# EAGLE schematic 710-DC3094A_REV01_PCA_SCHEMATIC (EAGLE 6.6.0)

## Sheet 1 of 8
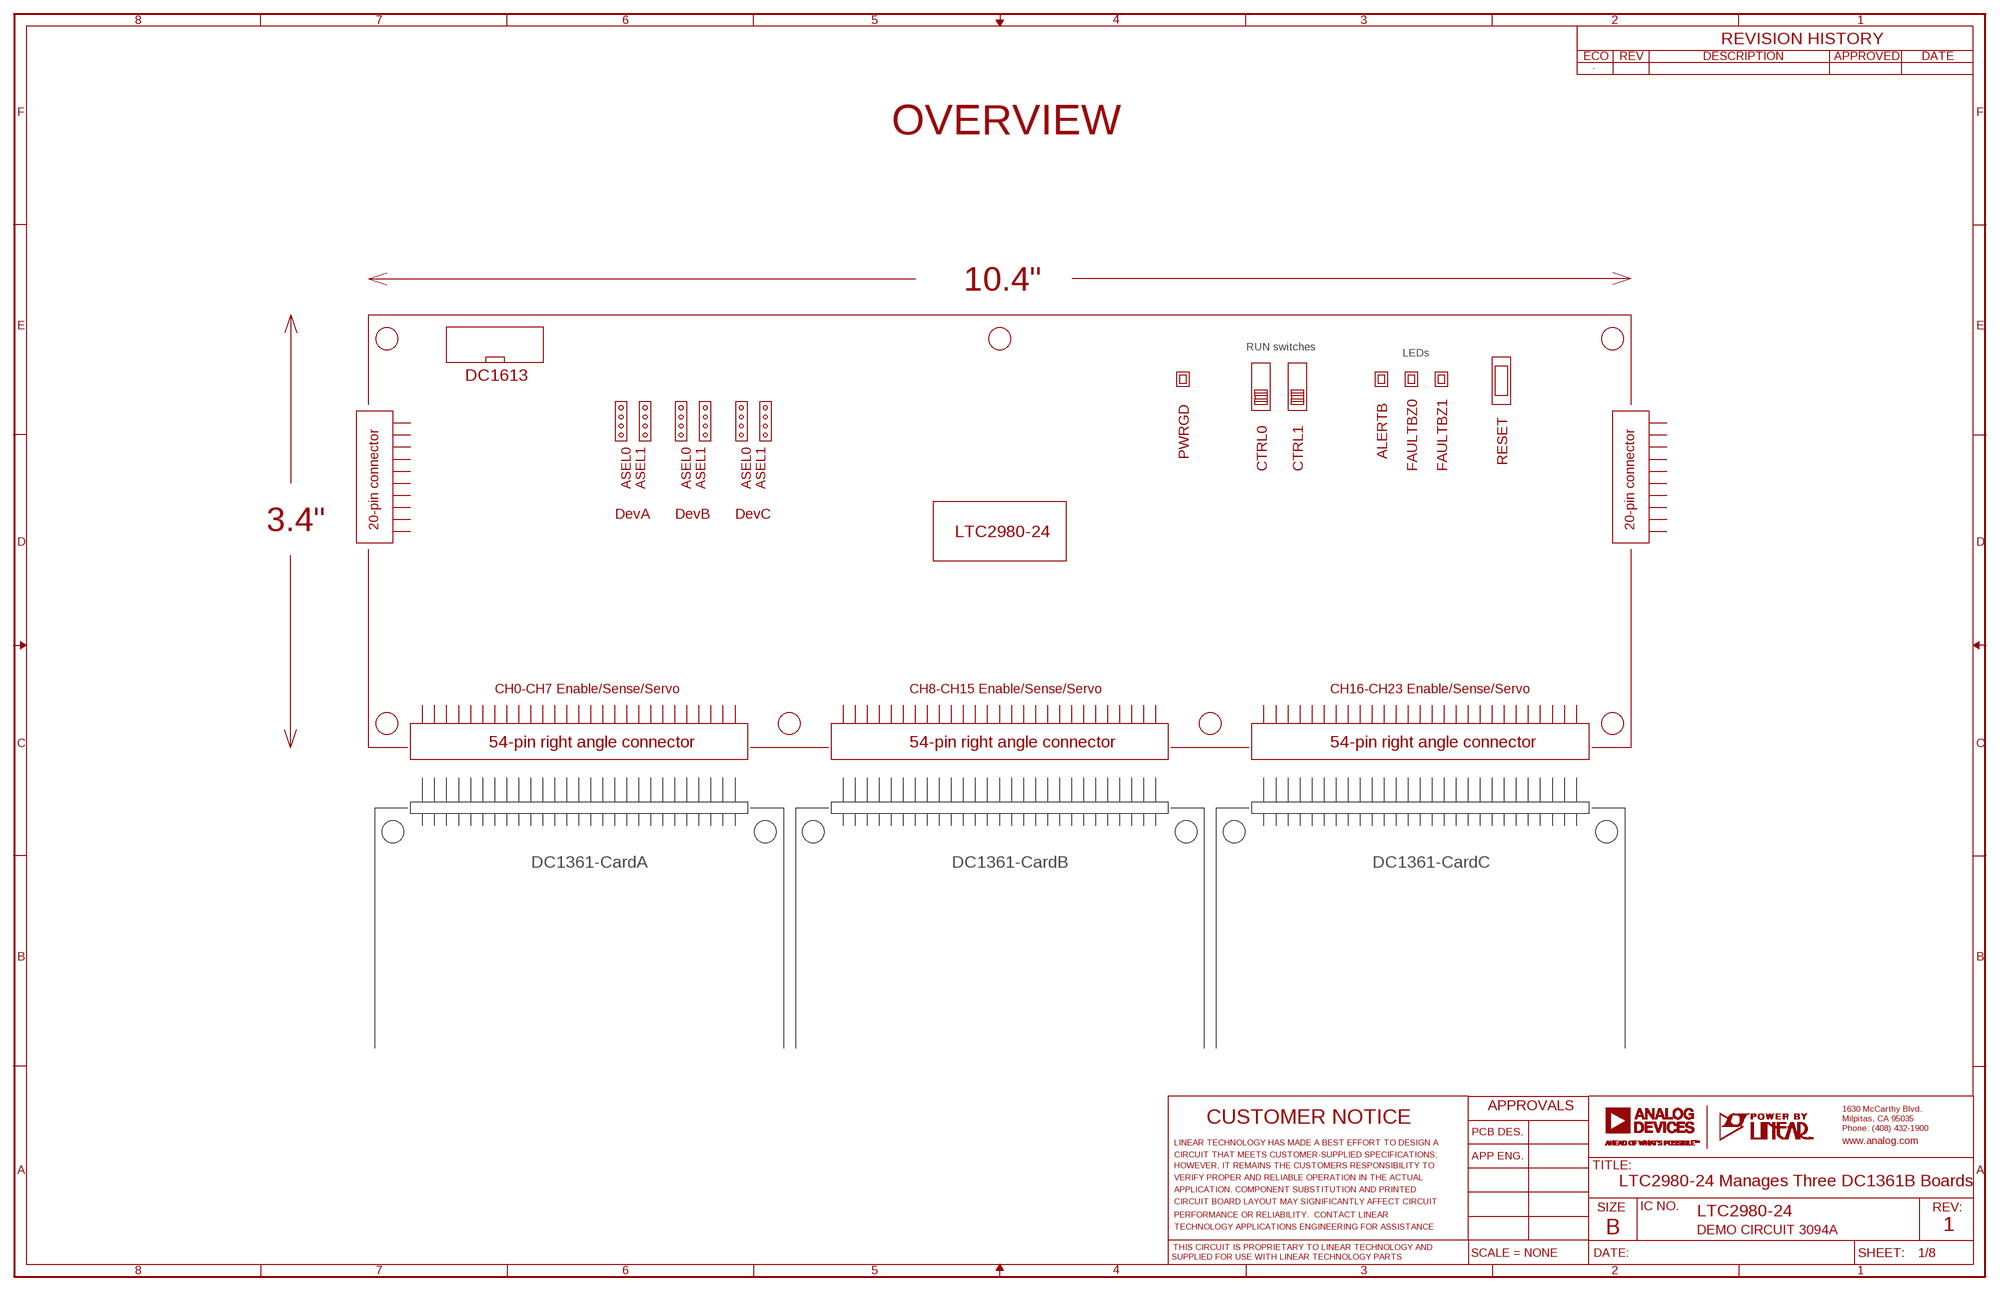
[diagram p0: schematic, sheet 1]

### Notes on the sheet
- OVERVIEW
- 10.4"
- RUN switches
- LEDs
- DC1613
- 20-pin connector | 20-pin connector
- ASEL0
  ASEL1
- ASEL0
  ASEL1
- ASEL0
  ASEL1
- PWRGD | ALERTB
- RESET
- CTRL0 | CTRL1 | FAULTBZ0 | FAULTBZ1
- DevA | DevB | DevC
- 3.4"
- LTC2980-24
- CH0-CH7 Enable/Sense/Servo | CH8-CH15 Enable/Sense/Servo | CH16-CH23 Enable/Sense/Servo
- 54-pin right angle connector | 54-pin right angle connector | 54-pin right angle connector
- DC1361-CardA | DC1361-CardB | DC1361-CardC
- LTC2980-24 Manages Three DC1361B Boards
- LTC2980-24
- DEMO CIRCUIT 3094A | 1

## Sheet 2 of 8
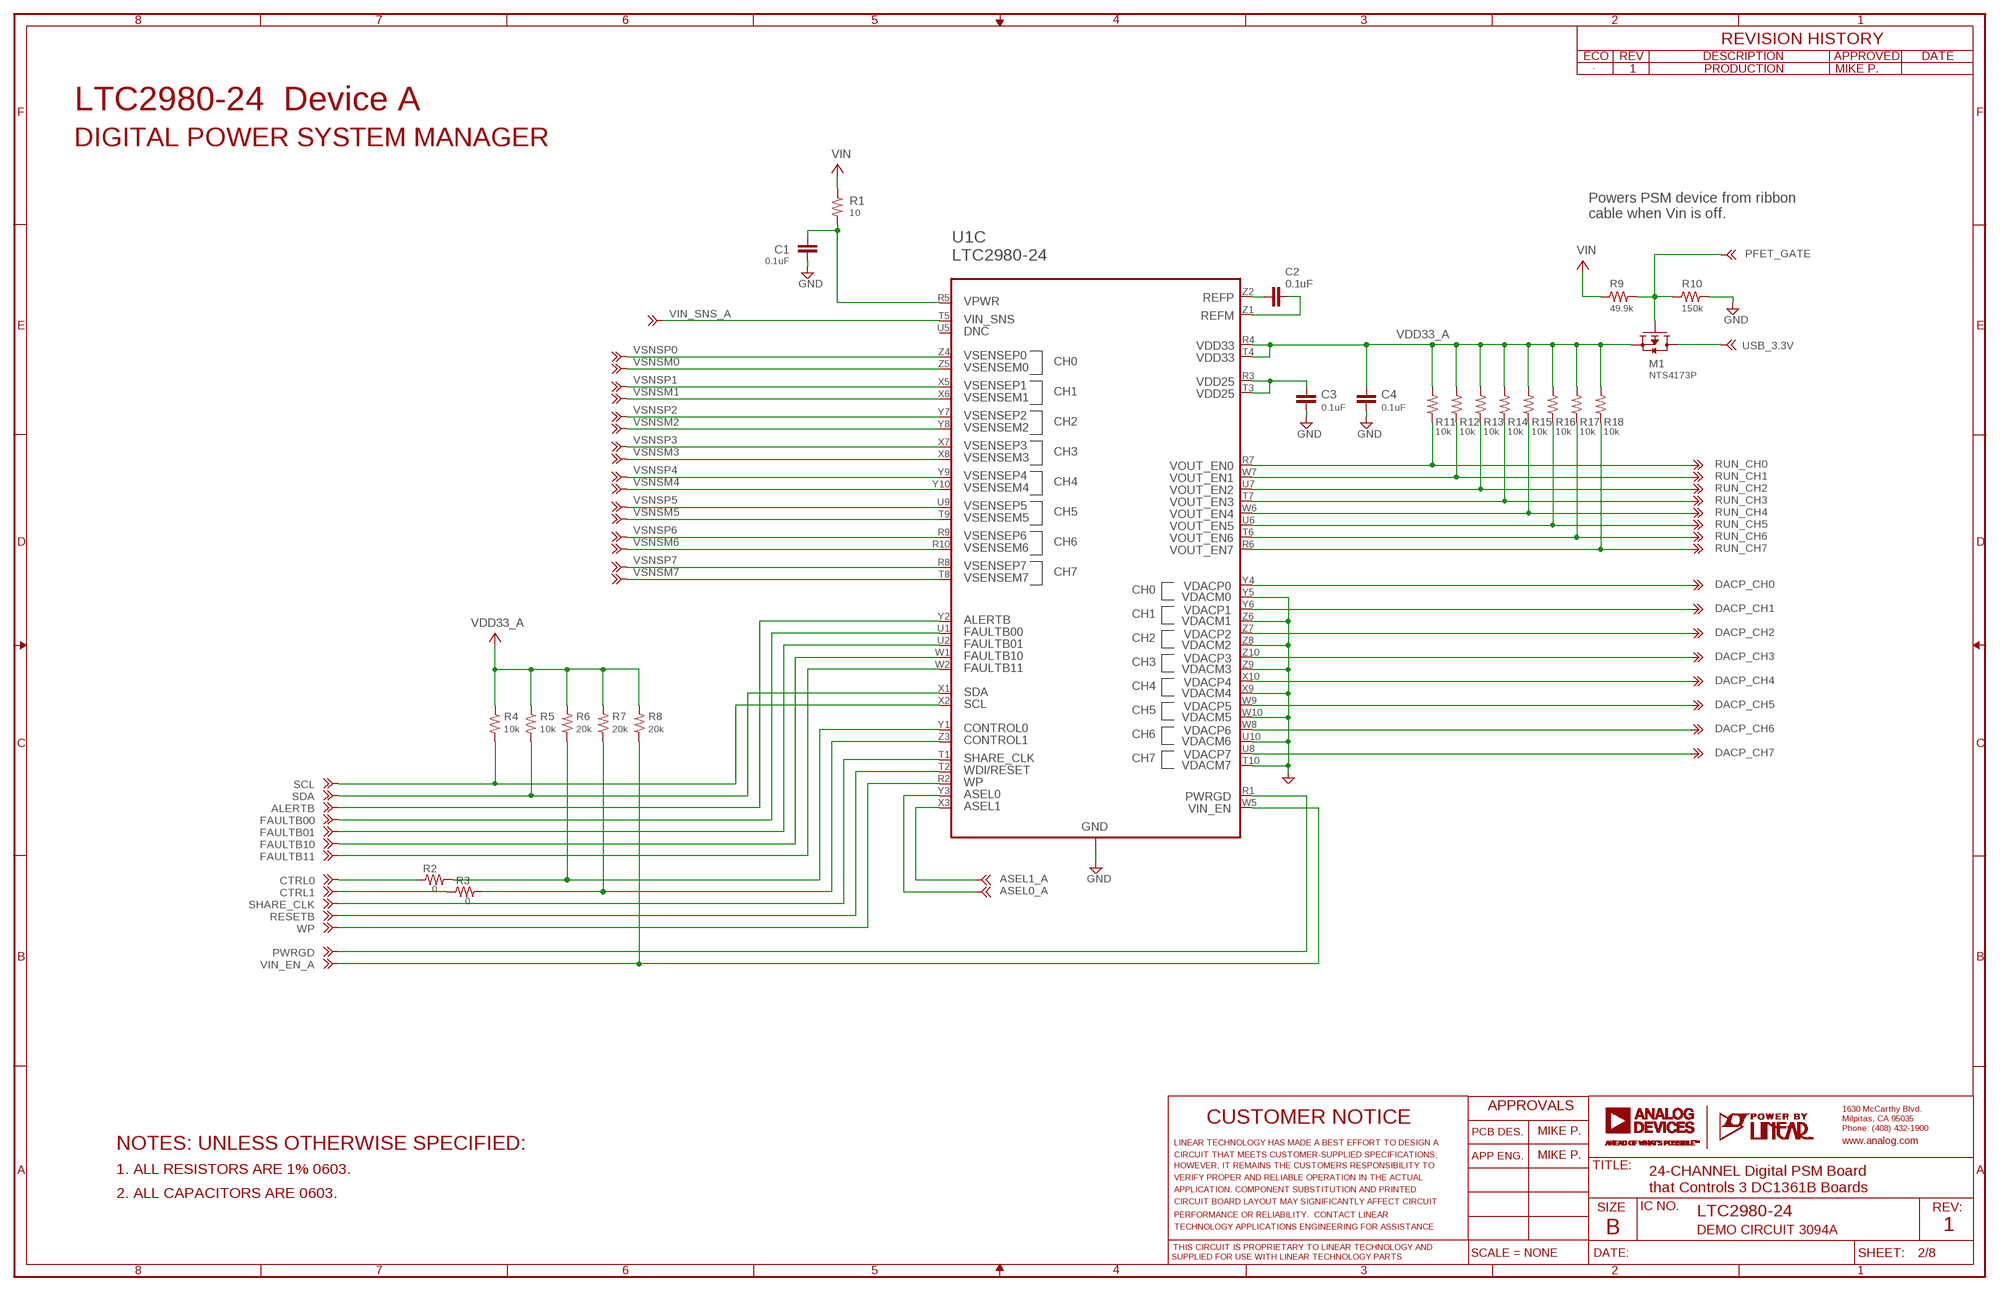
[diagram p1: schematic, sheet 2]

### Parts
C1  0.1uF  CC0603_BOX  [C0603_BOX]
C2  0.1uF  CC0603_BOX  [C0603_BOX]
C3  0.1uF  CC0603_BOX  [C0603_BOX]
C4  0.1uF  CC0603_BOX  [C0603_BOX]
M1  NTS4173P  PCH_SOT323  [SOT323@1]
R1  10  RR0603_BOX  [R0603_BOX]
R2  0  RR0603_BOX  [R0603_BOX]
R3  0  RR0603_BOX  [R0603_BOX]
R4  10k  RR0603_BOX  [R0603_BOX]
R5  10k  RR0603_BOX  [R0603_BOX]
R6  20k  RR0603_BOX  [R0603_BOX]
R7  20k  RR0603_BOX  [R0603_BOX]
R8  20k  RR0603_BOX  [R0603_BOX]
R9  49.9k  RR0402_BOX  [R0402_BOX]
R10  150k  RR0402_BOX  [R0402_BOX]
R11  10k  RR0603_BOX  [R0603_BOX]
R12  10k  RR0603_BOX  [R0603_BOX]
R13  10k  RR0603_BOX  [R0603_BOX]
R14  10k  RR0603_BOX  [R0603_BOX]
R15  10k  RR0603_BOX  [R0603_BOX]
R16  10k  RR0603_BOX  [R0603_BOX]
R17  10k  RR0603_BOX  [R0603_BOX]
R18  10k  RR0603_BOX  [R0603_BOX]
U1  LTC2980-24  LTC2980-24X  [BGA210]

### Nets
ALERTB: U1.Y2(C:ALERT) ; also sheet 3,4,5,8
ASEL0_A: U1.Y3(C:ASEL0) ; also sheet 5
ASEL1_A: U1.X3(C:ASEL1) ; also sheet 5
CTRL0: R2.1 ; also sheet 3,4,5,8
CTRL0_C: R2.2 R6.1 U1.Y1(C:CTRL0)
CTRL1: R3.1 ; also sheet 3,4,5,8
CTRL1_C: R3.2 R7.1 U1.Z3(C:CTRL1)
DACP_CH0: U1.Y4(C:DACP0) ; also sheet 7
DACP_CH1: U1.Y6(C:DACP1) ; also sheet 7
DACP_CH2: U1.Z7(C:DACP2) ; also sheet 7
DACP_CH3: U1.Z10(C:DACP3) ; also sheet 7
DACP_CH4: U1.X10(C:DACP4) ; also sheet 7
DACP_CH5: U1.W9(C:DACP5) ; also sheet 7
DACP_CH6: U1.W8(C:DACP6) ; also sheet 7
DACP_CH7: U1.U8(C:DACP7) ; also sheet 7
FAULTB00: U1.U1(C:FLT00) ; also sheet 3,4,5,8
FAULTB01: U1.U2(C:FLT01) ; also sheet 3,4,5,8
FAULTB10: U1.W1(C:FLT10) ; also sheet 3,4,5,8
FAULTB11: U1.W2(C:FLT11) ; also sheet 3,4,5,8
GND: C1.2 C3.2 C4.2 R10.2 U1.T10(C:DACM7) U1.U3(C:GND) U1.U4(C:GND) U1.U10(C:DACM6) U1.W3(C:GND) U1.W4(C:GND) U1.W10(C:DACM5) U1.X4(C:GND) U1.X9(C:DACM4) U1.Y5(C:DACM0) U1.Z6(C:DACM1) U1.Z8(C:DACM2) U1.Z9(C:DACM3) ; also sheet 3,4,5,6,7,8
PFET_GATE: M1.1(G) R9.2 R10.1 ; also sheet 3,4
PWRGD: U1.R1(C:PWRGD) ; also sheet 3,4,5
REFM_C: C2.2 U1.Z1(C:REFM)
REFP_C: C2.1 U1.Z2(C:REFP)
RESETB: U1.T2(C:WDI) ; also sheet 3,4,5,8
RUN_CH0: R11.1 U1.R7(C:EN0) ; also sheet 7
RUN_CH1: R12.1 U1.W7(C:EN1) ; also sheet 7
RUN_CH2: R13.1 U1.U7(C:EN2) ; also sheet 7
RUN_CH3: R14.1 U1.T7(C:EN3) ; also sheet 7
RUN_CH4: R15.1 U1.W6(C:EN4) ; also sheet 7
RUN_CH5: R16.1 U1.U6(C:EN5) ; also sheet 7
RUN_CH6: R17.1 U1.T6(C:EN6) ; also sheet 7
RUN_CH7: R18.1 U1.R6(C:EN7) ; also sheet 7
SCL: R4.2 U1.X2(C:SCL) ; also sheet 3,4,8
SDA: R5.2 U1.X1(C:SDA) ; also sheet 3,4,8
SHARE_CLK: U1.T1(C:SHARE_CLK) ; also sheet 3,4,8
USB_3.3V: M1.3(D) ; also sheet 3,4,8
VDD25_C: C3.1 U1.R3(C:VDD25-IN) U1.T3(C:VDD25-OUT)
VDD33_A: C4.1 M1.2(S) R4.1 R5.1 R6.2 R7.2 R8.2 R11.2 R12.2 R13.2 R14.2 R15.2 R16.2 R17.2 R18.2 U1.R4(C:VDD33-IN) U1.T4(C:VDD33-OUT) ; also sheet 5
VIN: R1.1 R9.1 ; also sheet 3,4,7
VIN_A: C1.1 R1.2 U1.R5(C:VPWR)
VIN_EN_A: R8.1 U1.W5(C:VINEN) ; also sheet 7,8
VIN_SNS_A: U1.T5(C:VINSNS) ; also sheet 7,8
VSNSM0: U1.Z5(C:VSM0) ; also sheet 6
VSNSM1: U1.X6(C:VSM1) ; also sheet 6
VSNSM2: U1.Y8(C:VSM2) ; also sheet 6
VSNSM3: U1.X8(C:VSM3) ; also sheet 6
VSNSM4: U1.Y10(C:VSM4) ; also sheet 6
VSNSM5: U1.T9(C:VSM5) ; also sheet 6
VSNSM6: U1.R10(C:VSM6) ; also sheet 6
VSNSM7: U1.T8(C:VSM7) ; also sheet 6
VSNSP0: U1.Z4(C:VSP0) ; also sheet 6
VSNSP1: U1.X5(C:VSP1) ; also sheet 6
VSNSP2: U1.Y7(C:VSP2) ; also sheet 6
VSNSP3: U1.X7(C:VSP3) ; also sheet 6
VSNSP4: U1.Y9(C:VSP4) ; also sheet 6
VSNSP5: U1.U9(C:VSP5) ; also sheet 6
VSNSP6: U1.R9(C:VSP6) ; also sheet 6
VSNSP7: U1.R8(C:VSP7) ; also sheet 6
WP: U1.R2(C:WP) ; also sheet 3,4,5
Unconnected: U1.U5(C:DNC)

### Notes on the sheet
- 1 | PRODUCTION | MIKE P.
- LTC2980-24  Device A
- DIGITAL POWER SYSTEM MANAGER
- Powers PSM device from ribbon
  cable when Vin is off.
- MIKE P.
- NOTES: UNLESS OTHERWISE SPECIFIED:
- MIKE P.
- 1. ALL RESISTORS ARE 1% 0603.
- 24-CHANNEL Digital PSM Board
  that Controls 3 DC1361B Boards
- 2. ALL CAPACITORS ARE 0603.
- LTC2980-24
- DEMO CIRCUIT 3094A | 1

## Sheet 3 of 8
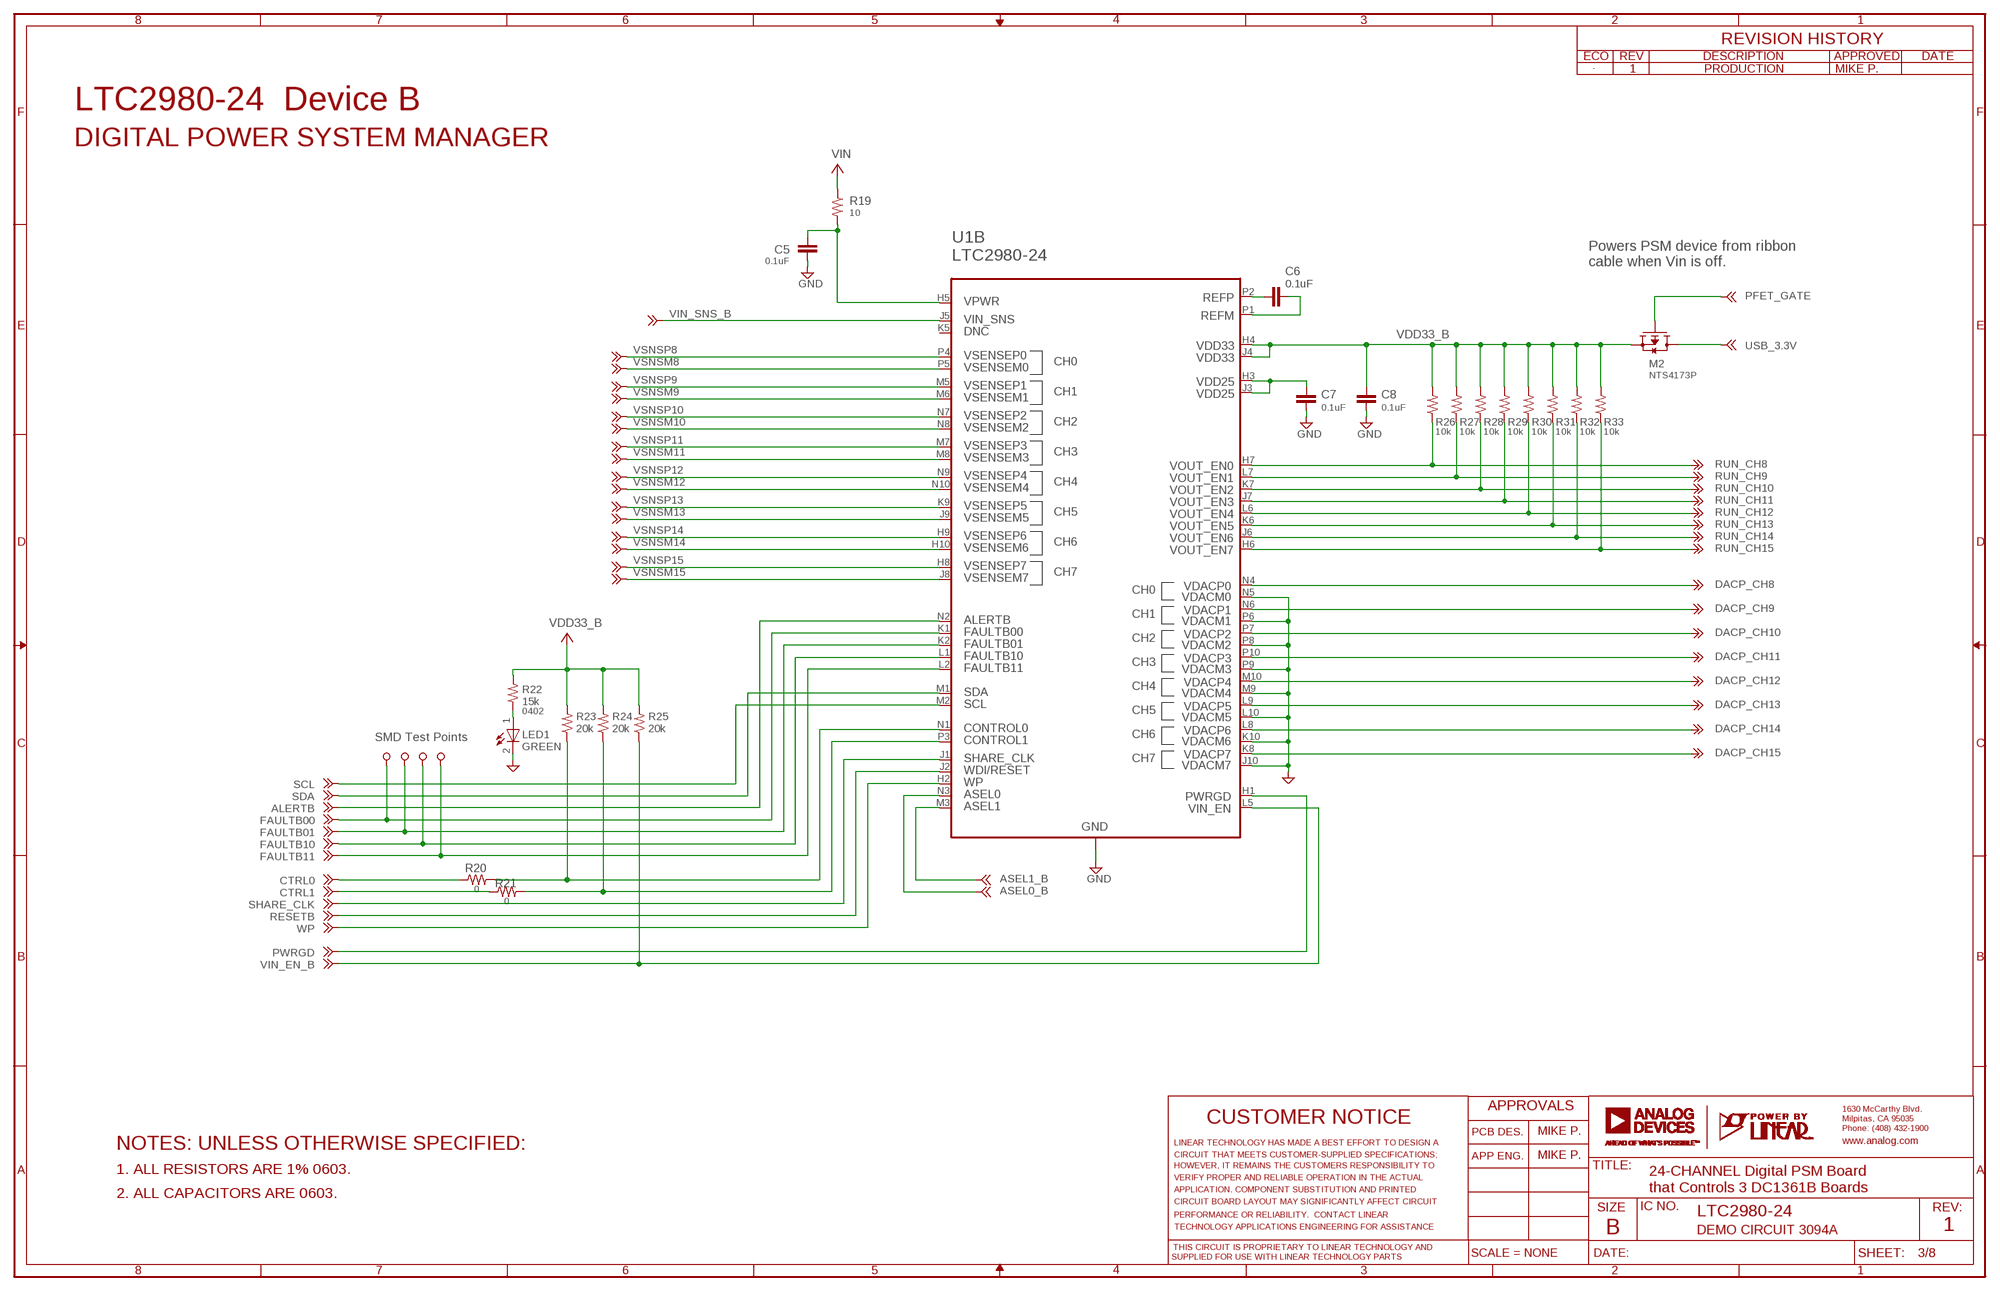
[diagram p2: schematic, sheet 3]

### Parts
C5  0.1uF  CC0603_BOX  [C0603_BOX]
C6  0.1uF  CC0603_BOX  [C0603_BOX]
C7  0.1uF  CC0603_BOX  [C0603_BOX]
C8  0.1uF  CC0603_BOX  [C0603_BOX]
LED1  GREEN  LED-0603  [CHIPLED_0603]
M2  NTS4173P  PCH_SOT323  [SOT323@1]
R19  10  RR0603_BOX  [R0603_BOX]
R20  0  RR0603_BOX  [R0603_BOX]
R21  0  RR0603_BOX  [R0603_BOX]
R22  15k  RR0402_BOX  [R0402_BOX]
R23  20k  RR0603_BOX  [R0603_BOX]
R24  20k  RR0603_BOX  [R0603_BOX]
R25  20k  RR0603_BOX  [R0603_BOX]
R26  10k  RR0603_BOX  [R0603_BOX]
R27  10k  RR0603_BOX  [R0603_BOX]
R28  10k  RR0603_BOX  [R0603_BOX]
R29  10k  RR0603_BOX  [R0603_BOX]
R30  10k  RR0603_BOX  [R0603_BOX]
R31  10k  RR0603_BOX  [R0603_BOX]
R32  10k  RR0603_BOX  [R0603_BOX]
R33  10k  RR0603_BOX  [R0603_BOX]
TP10  TESTPOINTVIA  [VIA]
TP11  TESTPOINTVIA  [VIA]
TP12  TESTPOINTVIA  [VIA]
TP13  TESTPOINTVIA  [VIA]

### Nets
ALERTB: U1.N2(B:ALERT) ; also sheet 2,4,5,8
ASEL0_B: U1.N3(B:ASEL0) ; also sheet 5
ASEL1_B: U1.M3(B:ASEL1) ; also sheet 5
CTRL0: R20.1 ; also sheet 2,4,5,8
CTRL0_B: R20.2 R23.1 U1.N1(B:CTRL0)
CTRL1: R21.1 ; also sheet 2,4,5,8
CTRL1_B: R21.2 R24.1 U1.P3(B:CTRL1)
DACP_CH8: U1.N4(B:DACP0) ; also sheet 7
DACP_CH9: U1.N6(B:DACP1) ; also sheet 7
DACP_CH10: U1.P7(B:DACP2) ; also sheet 7
DACP_CH11: U1.P10(B:DACP3) ; also sheet 7
DACP_CH12: U1.M10(B:DACP4) ; also sheet 7
DACP_CH13: U1.L9(B:DACP5) ; also sheet 7
DACP_CH14: U1.L8(B:DACP6) ; also sheet 7
DACP_CH15: U1.K8(B:DACP7) ; also sheet 7
FAULTB00: TP10.1 U1.K1(B:FLT00) ; also sheet 2,4,5,8
FAULTB01: TP11.1 U1.K2(B:FLT01) ; also sheet 2,4,5,8
FAULTB10: TP12.1 U1.L1(B:FLT10) ; also sheet 2,4,5,8
FAULTB11: TP13.1 U1.L2(B:FLT11) ; also sheet 2,4,5,8
GND: C5.2 C7.2 C8.2 LED1.N(C) U1.J10(B:DACM7) U1.K3(B:GND) U1.K4(B:GND) U1.K10(B:DACM6) U1.L3(B:GND) U1.L4(B:GND) U1.L10(B:DACM5) U1.M4(B:GND) U1.M9(B:DACM4) U1.N5(B:DACM0) U1.P6(B:DACM1) U1.P8(B:DACM2) U1.P9(B:DACM3) ; also sheet 2,4,5,6,7,8
N$4: LED1.P(A) R22.1
PFET_GATE: M2.1(G) ; also sheet 2,4
PWRGD: U1.H1(B:PWRGD) ; also sheet 2,4,5
REFM_B: C6.2 U1.P1(B:REFM)
REFP_B: C6.1 U1.P2(B:REFP)
RESETB: U1.J2(B:WDI) ; also sheet 2,4,5,8
RUN_CH8: R26.1 U1.H7(B:EN0) ; also sheet 7
RUN_CH9: R27.1 U1.L7(B:EN1) ; also sheet 7
RUN_CH10: R28.1 U1.K7(B:EN2) ; also sheet 7
RUN_CH11: R29.1 U1.J7(B:EN3) ; also sheet 7
RUN_CH12: R30.1 U1.L6(B:EN4) ; also sheet 7
RUN_CH13: R31.1 U1.K6(B:EN5) ; also sheet 7
RUN_CH14: R32.1 U1.J6(B:EN6) ; also sheet 7
RUN_CH15: R33.1 U1.H6(B:EN7) ; also sheet 7
SCL: U1.M2(B:SCL) ; also sheet 2,4,8
SDA: U1.M1(B:SDA) ; also sheet 2,4,8
SHARE_CLK: U1.J1(B:SHARE_CLK) ; also sheet 2,4,8
USB_3.3V: M2.3(D) ; also sheet 2,4,8
VDD25_B: C7.1 U1.H3(B:VDD25-IN) U1.J3(B:VDD25-OUT)
VDD33_B: C8.1 M2.2(S) R22.2 R23.2 R24.2 R25.2 R26.2 R27.2 R28.2 R29.2 R30.2 R31.2 R32.2 R33.2 U1.H4(B:VDD33-IN) U1.J4(B:VDD33-OUT) ; also sheet 5
VIN: R19.1 ; also sheet 2,4,7
VIN_B: C5.1 R19.2 U1.H5(B:VPWR)
VIN_EN_B: R25.1 U1.L5(B:VINEN) ; also sheet 7,8
VIN_SNS_B: U1.J5(B:VINSNS) ; also sheet 7,8
VSNSM8: U1.P5(B:VSM0) ; also sheet 6
VSNSM9: U1.M6(B:VSM1) ; also sheet 6
VSNSM10: U1.N8(B:VSM2) ; also sheet 6
VSNSM11: U1.M8(B:VSM3) ; also sheet 6
VSNSM12: U1.N10(B:VSM4) ; also sheet 6
VSNSM13: U1.J9(B:VSM5) ; also sheet 6
VSNSM14: U1.H10(B:VSM6) ; also sheet 6
VSNSM15: U1.J8(B:VSM7) ; also sheet 6
VSNSP8: U1.P4(B:VSP0) ; also sheet 6
VSNSP9: U1.M5(B:VSP1) ; also sheet 6
VSNSP10: U1.N7(B:VSP2) ; also sheet 6
VSNSP11: U1.M7(B:VSP3) ; also sheet 6
VSNSP12: U1.N9(B:VSP4) ; also sheet 6
VSNSP13: U1.K9(B:VSP5) ; also sheet 6
VSNSP14: U1.H9(B:VSP6) ; also sheet 6
VSNSP15: U1.H8(B:VSP7) ; also sheet 6
WP: U1.H2(B:WP) ; also sheet 2,4,5
Unconnected: U1.K5(B:DNC)

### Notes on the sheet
- 1 | PRODUCTION | MIKE P.
- LTC2980-24  Device B
- DIGITAL POWER SYSTEM MANAGER
- Powers PSM device from ribbon
  cable when Vin is off.
- 0402
- SMD Test Points
- MIKE P.
- NOTES: UNLESS OTHERWISE SPECIFIED:
- MIKE P.
- 1. ALL RESISTORS ARE 1% 0603.
- 24-CHANNEL Digital PSM Board
  that Controls 3 DC1361B Boards
- 2. ALL CAPACITORS ARE 0603.
- LTC2980-24
- DEMO CIRCUIT 3094A | 1

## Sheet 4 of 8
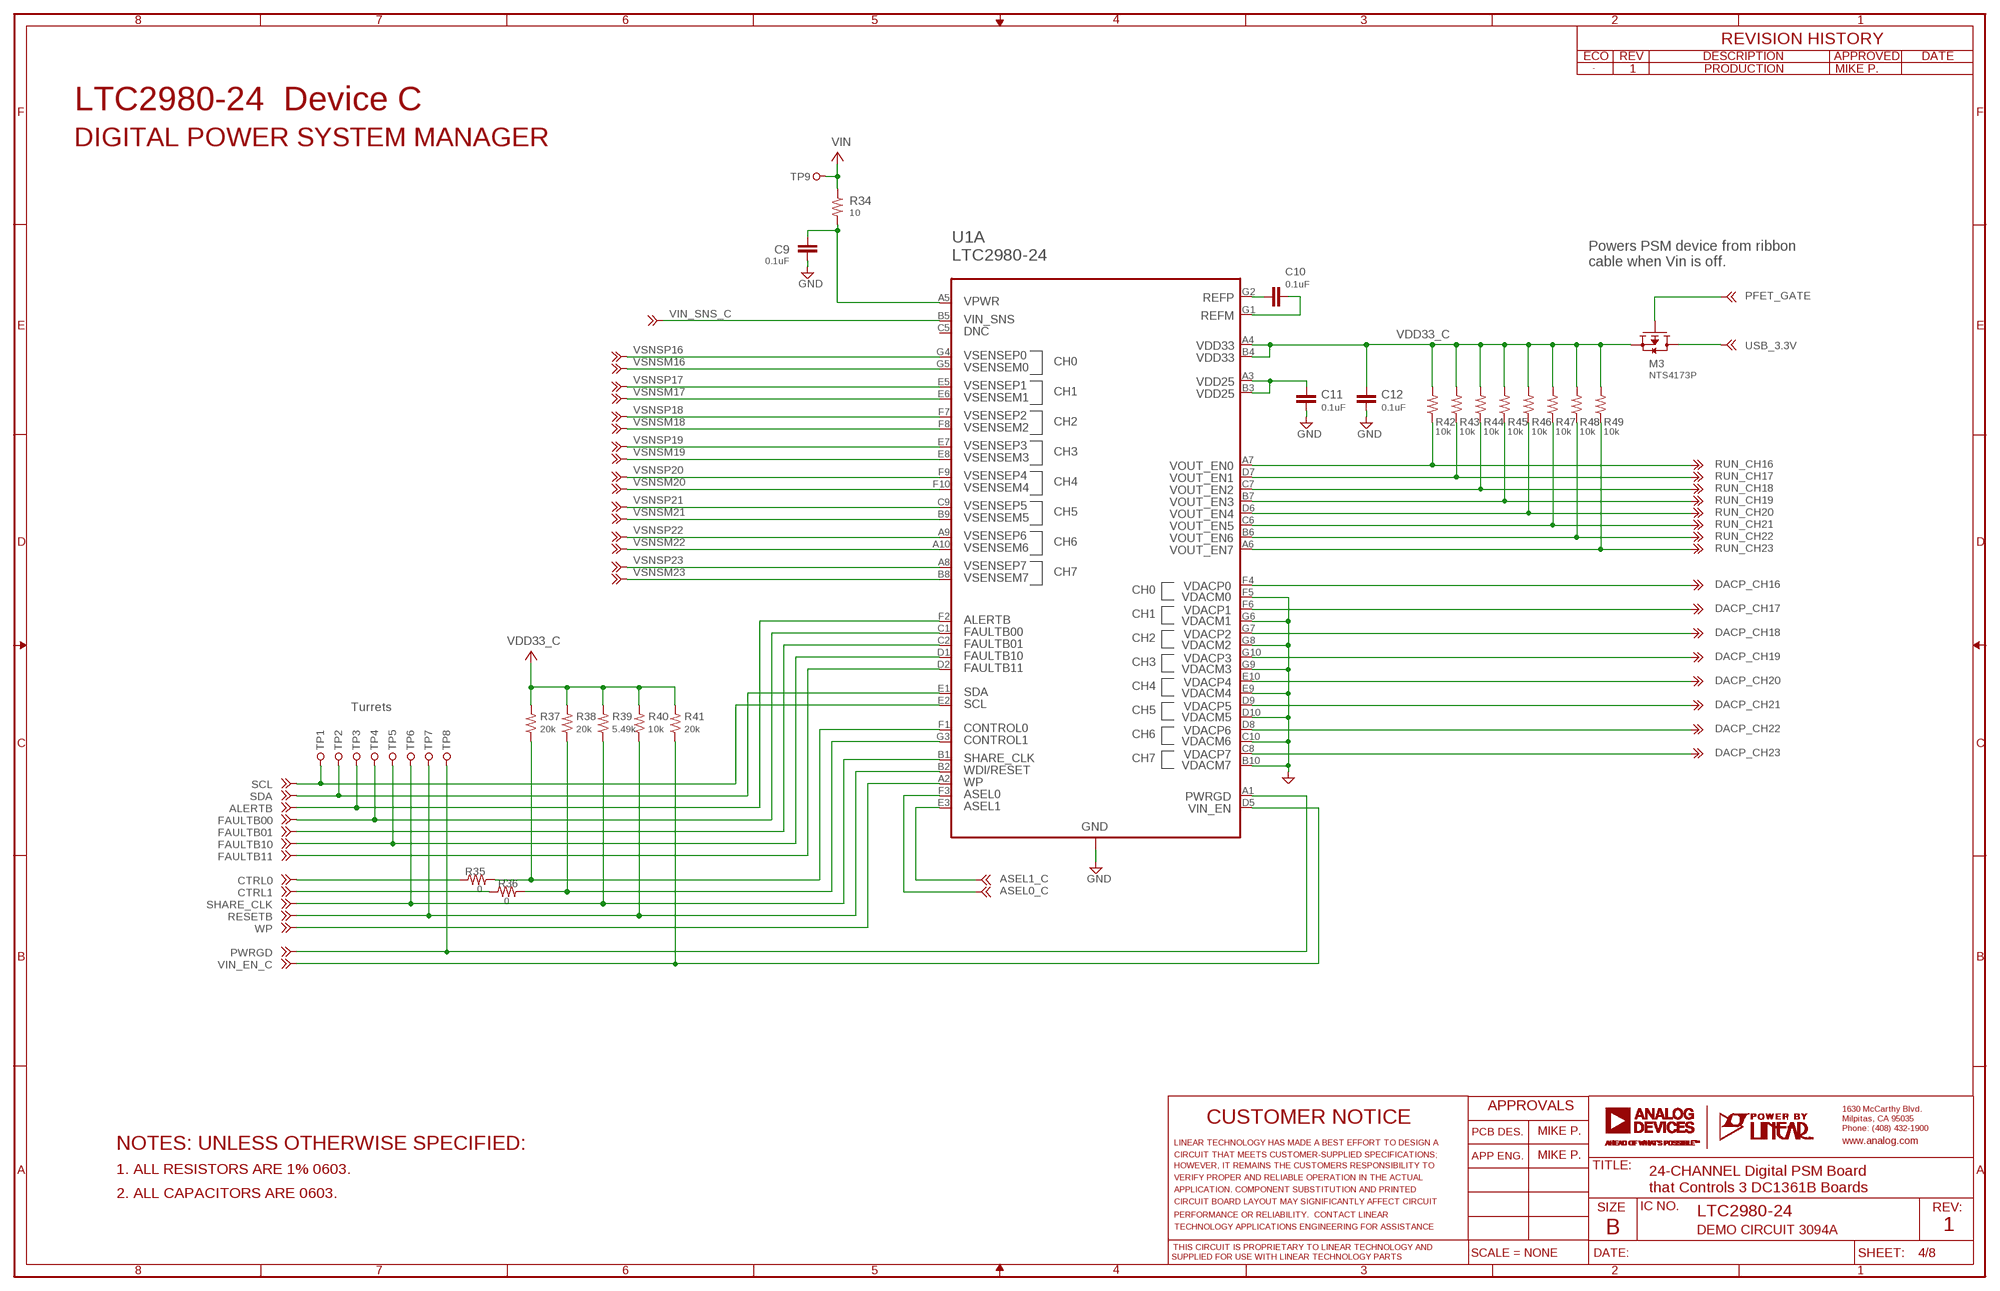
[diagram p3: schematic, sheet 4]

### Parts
C9  0.1uF  CC0603_BOX  [C0603_BOX]
C10  0.1uF  CC0603_BOX  [C0603_BOX]
C11  0.1uF  CC0603_BOX  [C0603_BOX]
C12  0.1uF  CC0603_BOX  [C0603_BOX]
M3  NTS4173P  PCH_SOT323  [SOT323@1]
R34  10  RR0603_BOX  [R0603_BOX]
R35  0  RR0603_BOX  [R0603_BOX]
R36  0  RR0603_BOX  [R0603_BOX]
R37  20k  RR0603_BOX  [R0603_BOX]
R38  20k  RR0603_BOX  [R0603_BOX]
R39  5.49k  RR0603_BOX  [R0603_BOX]
R40  10k  RR0603_BOX  [R0603_BOX]
R41  20k  RR0603_BOX  [R0603_BOX]
R42  10k  RR0603_BOX  [R0603_BOX]
R43  10k  RR0603_BOX  [R0603_BOX]
R44  10k  RR0603_BOX  [R0603_BOX]
R45  10k  RR0603_BOX  [R0603_BOX]
R46  10k  RR0603_BOX  [R0603_BOX]
R47  10k  RR0603_BOX  [R0603_BOX]
R48  10k  RR0603_BOX  [R0603_BOX]
R49  10k  RR0603_BOX  [R0603_BOX]
TP1  TURRET_LARGE_2501  [TURRET_LARGE_2501]
TP2  TURRET_LARGE_2501  [TURRET_LARGE_2501]
TP3  TURRET_LARGE_2501  [TURRET_LARGE_2501]
TP4  TURRET_LARGE_2501  [TURRET_LARGE_2501]
TP5  TURRET_LARGE_2501  [TURRET_LARGE_2501]
TP6  TURRET_LARGE_2501  [TURRET_LARGE_2501]
TP7  TURRET_LARGE_2501  [TURRET_LARGE_2501]
TP8  TURRET_LARGE_2501  [TURRET_LARGE_2501]
TP9  TURRET_LARGE_2501  [TURRET_LARGE_2501]

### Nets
ALERTB: TP3.TP U1.F2(A:ALERT) ; also sheet 2,3,5,8
ASEL0_C: U1.F3(A:ASEL0) ; also sheet 5
ASEL1_C: U1.E3(A:ASEL1) ; also sheet 5
CTRL0: R35.1 ; also sheet 2,3,5,8
CTRL0_A: R35.2 R37.1 U1.F1(A:CTRL0)
CTRL1: R36.1 ; also sheet 2,3,5,8
CTRL1_A: R36.2 R38.1 U1.G3(A:CTRL1)
DACP_CH16: U1.F4(A:DACP0) ; also sheet 7
DACP_CH17: U1.F6(A:DACP1) ; also sheet 7
DACP_CH18: U1.G7(A:DACP2) ; also sheet 7
DACP_CH19: U1.G10(A:DACP3) ; also sheet 7
DACP_CH20: U1.E10(A:DACP4) ; also sheet 7
DACP_CH21: U1.D9(A:DACP5) ; also sheet 7
DACP_CH22: U1.D8(A:DACP6) ; also sheet 7
DACP_CH23: U1.C8(A:DACP7) ; also sheet 7
FAULTB00: TP4.TP U1.C1(A:FLT00) ; also sheet 2,3,5,8
FAULTB01: U1.C2(A:FLT01) ; also sheet 2,3,5,8
FAULTB10: TP5.TP U1.D1(A:FLT10) ; also sheet 2,3,5,8
FAULTB11: U1.D2(A:FLT11) ; also sheet 2,3,5,8
GND: C9.2 C11.2 C12.2 U1.B10(A:DACM7) U1.C3(A:GND) U1.C4(A:GND) U1.C10(A:DACM6) U1.D3(A:GND) U1.D4(A:GND) U1.D10(A:DACM5) U1.E4(A:GND) U1.E9(A:DACM4) U1.F5(A:DACM0) U1.G6(A:DACM1) U1.G8(A:DACM2) U1.G9(A:DACM3) ; also sheet 2,3,5,6,7,8
PFET_GATE: M3.1(G) ; also sheet 2,3
PWRGD: TP8.TP U1.A1(A:PWRGD) ; also sheet 2,3,5
REFM_A: C10.2 U1.G1(A:REFM)
REFP_A: C10.1 U1.G2(A:REFP)
RESETB: R40.1 TP7.TP U1.B2(A:WDI) ; also sheet 2,3,5,8
RUN_CH16: R42.1 U1.A7(A:EN0) ; also sheet 7
RUN_CH17: R43.1 U1.D7(A:EN1) ; also sheet 7
RUN_CH18: R44.1 U1.C7(A:EN2) ; also sheet 7
RUN_CH19: R45.1 U1.B7(A:EN3) ; also sheet 7
RUN_CH20: R46.1 U1.D6(A:EN4) ; also sheet 7
RUN_CH21: R47.1 U1.C6(A:EN5) ; also sheet 7
RUN_CH22: R48.1 U1.B6(A:EN6) ; also sheet 7
RUN_CH23: R49.1 U1.A6(A:EN7) ; also sheet 7
SCL: TP1.TP U1.E2(A:SCL) ; also sheet 2,3,8
SDA: TP2.TP U1.E1(A:SDA) ; also sheet 2,3,8
SHARE_CLK: R39.1 TP6.TP U1.B1(A:SHARE_CLK) ; also sheet 2,3,8
USB_3.3V: M3.3(D) ; also sheet 2,3,8
VDD25_A: C11.1 U1.A3(A:VDD25-IN) U1.B3(A:VDD25-OUT)
VDD33_C: C12.1 M3.2(S) R37.2 R38.2 R39.2 R40.2 R41.2 R42.2 R43.2 R44.2 R45.2 R46.2 R47.2 R48.2 R49.2 U1.A4(A:VDD33-IN) U1.B4(A:VDD33-OUT) ; also sheet 5,8
VIN: R34.1 TP9.TP ; also sheet 2,3,7
VIN_C: C9.1 R34.2 U1.A5(A:VPWR)
VIN_EN_C: R41.1 U1.D5(A:VINEN) ; also sheet 7,8
VIN_SNS_C: U1.B5(A:VINSNS) ; also sheet 7,8
VSNSM16: U1.G5(A:VSM0) ; also sheet 6
VSNSM17: U1.E6(A:VSM1) ; also sheet 6
VSNSM18: U1.F8(A:VSM2) ; also sheet 6
VSNSM19: U1.E8(A:VSM3) ; also sheet 6
VSNSM20: U1.F10(A:VSM4) ; also sheet 6
VSNSM21: U1.B9(A:VSM5) ; also sheet 6
VSNSM22: U1.A10(A:VSM6) ; also sheet 6
VSNSM23: U1.B8(A:VSM7) ; also sheet 6
VSNSP16: U1.G4(A:VSP0) ; also sheet 6
VSNSP17: U1.E5(A:VSP1) ; also sheet 6
VSNSP18: U1.F7(A:VSP2) ; also sheet 6
VSNSP19: U1.E7(A:VSP3) ; also sheet 6
VSNSP20: U1.F9(A:VSP4) ; also sheet 6
VSNSP21: U1.C9(A:VSP5) ; also sheet 6
VSNSP22: U1.A9(A:VSP6) ; also sheet 6
VSNSP23: U1.A8(A:VSP7) ; also sheet 6
WP: U1.A2(A:WP) ; also sheet 2,3,5
Unconnected: U1.C5(A:DNC)

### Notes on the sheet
- 1 | PRODUCTION | MIKE P.
- LTC2980-24  Device C
- DIGITAL POWER SYSTEM MANAGER
- Powers PSM device from ribbon
  cable when Vin is off.
- Turrets
- MIKE P.
- NOTES: UNLESS OTHERWISE SPECIFIED:
- MIKE P.
- 1. ALL RESISTORS ARE 1% 0603.
- 24-CHANNEL Digital PSM Board
  that Controls 3 DC1361B Boards
- 2. ALL CAPACITORS ARE 0603.
- LTC2980-24
- DEMO CIRCUIT 3094A | 1

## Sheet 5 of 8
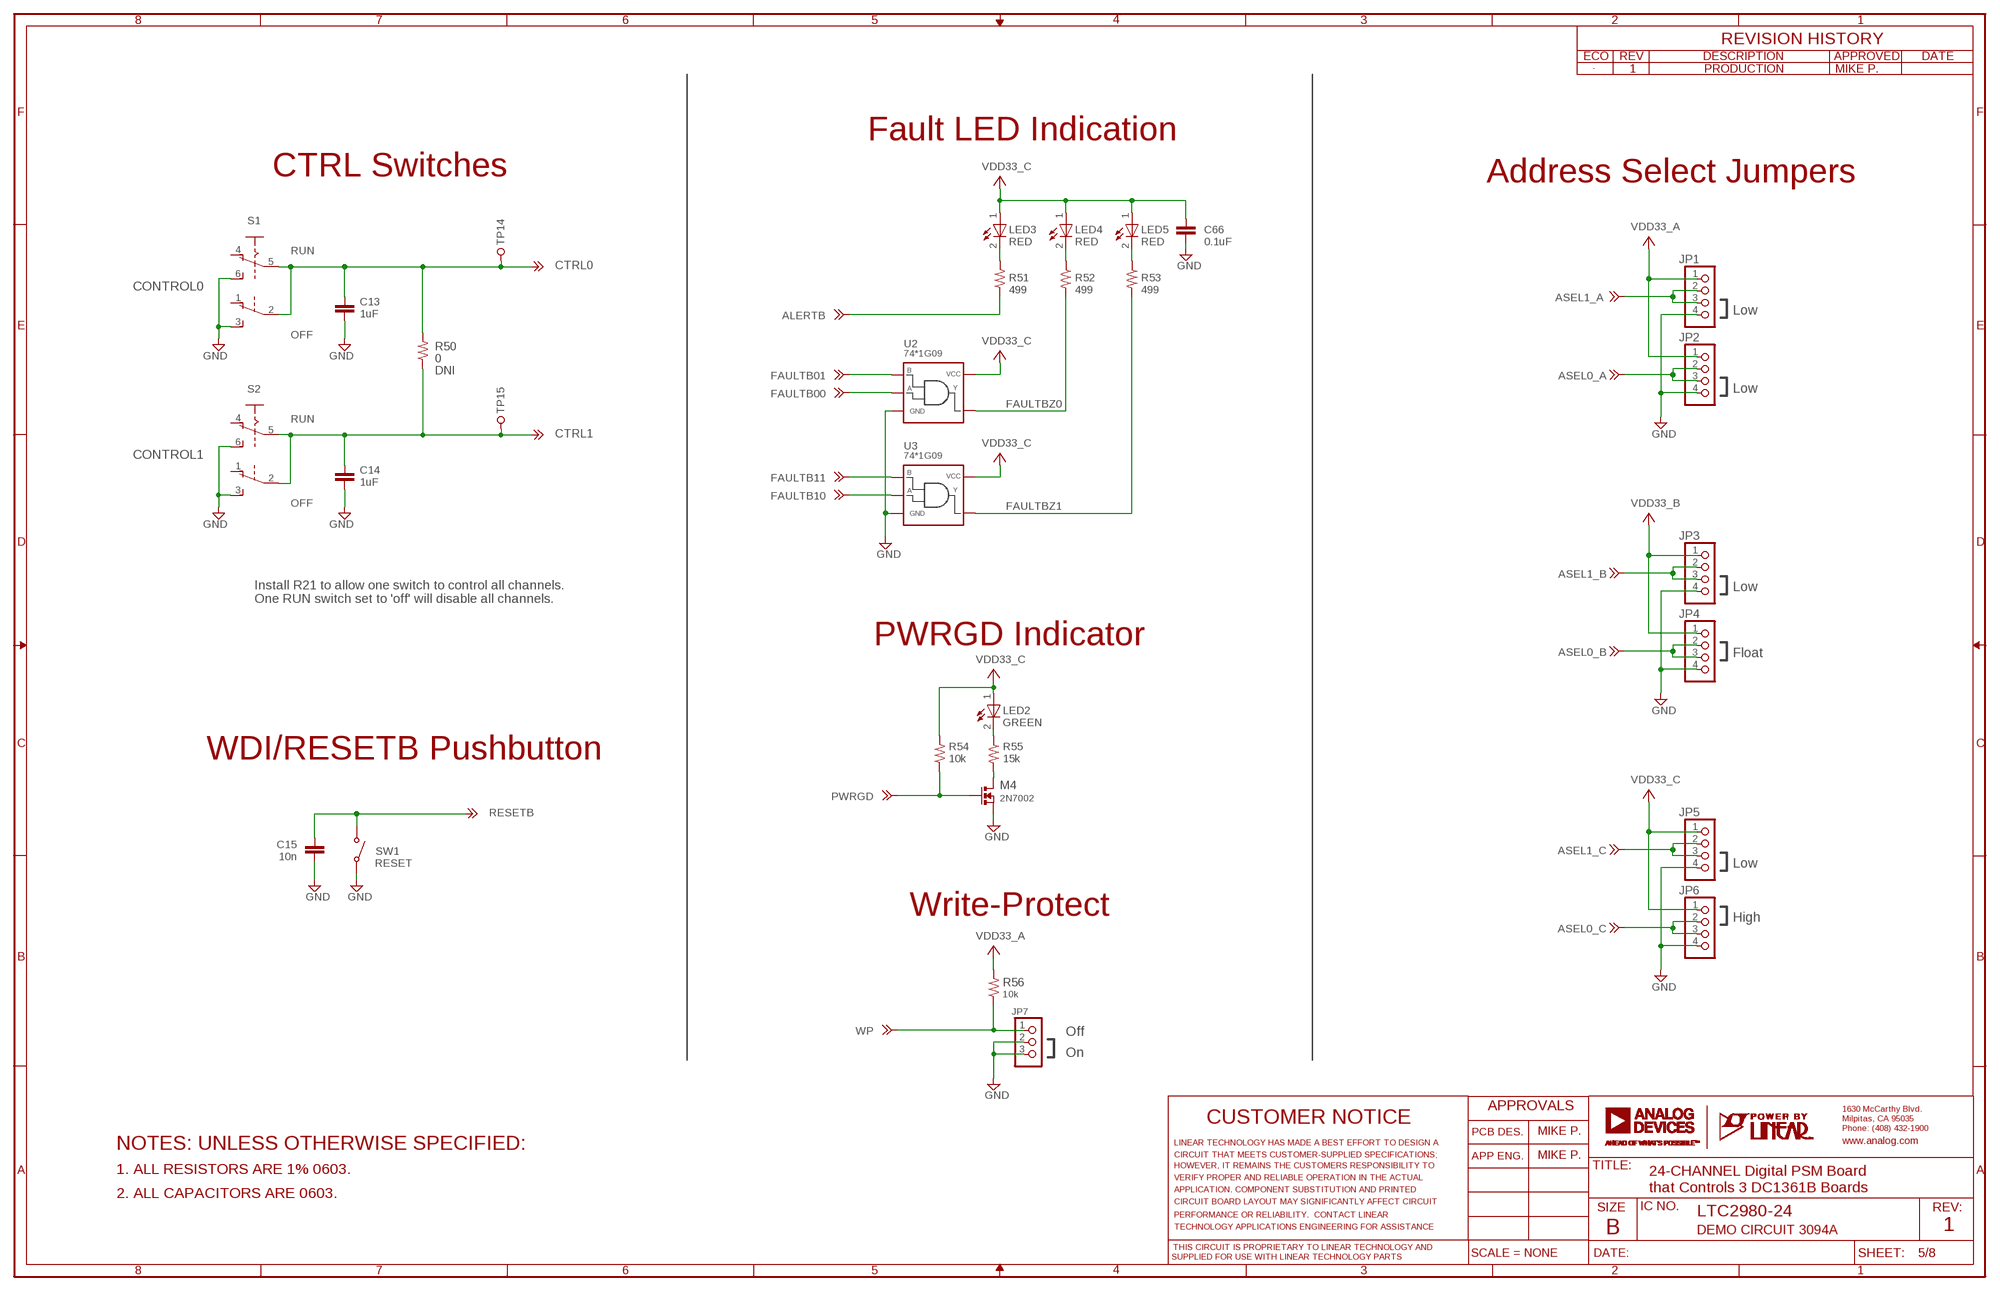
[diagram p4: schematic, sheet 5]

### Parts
C13  1uF  CC0603_BOX  [C0603_BOX]
C14  1uF  CC0603_BOX  [C0603_BOX]
C15  10n  CC0603_BOX  [C0603_BOX]
C66  0.1uF  CC0603_BOX  [C0603_BOX]
JP1  PINHD-1X4-2MM  [1X04-2MM]
JP2  PINHD-1X4-2MM  [1X04-2MM]
JP3  PINHD-1X4-2MM  [1X04-2MM]
JP4  PINHD-1X4-2MM  [1X04-2MM]
JP5  PINHD-1X4-2MM  [1X04-2MM]
JP6  PINHD-1X4-2MM  [1X04-2MM]
JP7  PINHD-1X3-2MM  [1X03-2MM]
LED2  GREEN  LED-0603  [CHIPLED_0603]
LED3  RED  LED-0603  [CHIPLED_0603]
LED4  RED  LED-0603  [CHIPLED_0603]
LED5  RED  LED-0603  [CHIPLED_0603]
M4  2N7002  NCH(SOT23)  [SOT23]
R50  0  RR0402_BOX  [R0402_BOX]
R51  499  RR0603_BOX  [R0603_BOX]
R52  499  RR0603_BOX  [R0603_BOX]
R53  499  RR0603_BOX  [R0603_BOX]
R54  10k  RR0603_BOX  [R0603_BOX]
R55  15k  RR0402_BOX  [R0402_BOX]
R56  10k  RR0603_BOX  [R0603_BOX]
S1  CONTROL0  JS202011CQN  [JS202011CQN]
S2  CONTROL1  JS202011CQN  [JS202011CQN]
SW1  PTS635SL25SMTR LFS  SWITCH_PTS635  [SWITCH_PTS635]
TP14  TURRET_LARGE_2501  [TURRET_LARGE_2501]
TP15  TURRET_LARGE_2501  [TURRET_LARGE_2501]
U2  74*1G09  741G09SOT23  [SOT23-5]
U3  74*1G09  741G09SOT23  [SOT23-5]

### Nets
ALERTB: R51.1 ; also sheet 2,3,4,8
ASEL0_A: JP2.2 JP2.3 ; also sheet 2
ASEL0_B: JP4.2 JP4.3 ; also sheet 3
ASEL0_C: JP6.2 JP6.3 ; also sheet 4
ASEL1_A: JP1.2 JP1.3 ; also sheet 2
ASEL1_B: JP3.2 JP3.3 ; also sheet 3
ASEL1_C: JP5.2 JP5.3 ; also sheet 4
CTRL0: C13.1 R50.2 S1.2(B:P) S1.5(A:P) TP14.TP ; also sheet 2,3,4,8
CTRL1: C14.1 R50.1 S2.2(B:P) S2.5(A:P) TP15.TP ; also sheet 2,3,4,8
FAULTB00: U2.2(A) ; also sheet 2,3,4,8
FAULTB01: U2.1(B) ; also sheet 2,3,4,8
FAULTB10: U3.2(A) ; also sheet 2,3,4,8
FAULTB11: U3.1(B) ; also sheet 2,3,4,8
FAULTBZ0: R52.2 U2.4(Y)
FAULTBZ1: R53.2 U3.4(Y)
GND: C13.2 C14.2 C15.1 C66.2 JP1.4 JP2.4 JP3.4 JP4.4 JP5.4 JP6.4 JP7.2 JP7.3 M4.2(S) S1.3(B:S) S1.6(A:S) S2.3(B:S) S2.6(A:S) SW1.SW2 U2.3(GND) U3.3(GND) ; also sheet 2,3,4,6,7,8
N$2: LED2.N(C) R55.1
N$8: M4.3(D) R55.2
N$28: LED5.N(C) R53.1
N$29: LED4.N(C) R52.1
N$30: LED3.N(C) R51.2
PWRGD: M4.1(G) R54.1 ; also sheet 2,3,4
RESETB: C15.2 SW1.SW1 ; also sheet 2,3,4,8
VDD33_A: JP1.1 JP2.1 R56.2 ; supply symbol labelled +3V3 ; also sheet 2
VDD33_B: JP3.1 JP4.1 ; supply symbol labelled +3V3 ; also sheet 3
VDD33_C: C66.1 JP5.1 JP6.1 LED2.P(A) LED3.P(A) LED4.P(A) LED5.P(A) R54.2 U2.5(VCC) U3.5(VCC) ; supply symbol labelled +3V3 ; also sheet 4,8
WP: JP7.1 R56.1 ; also sheet 2,3,4
Unconnected: S1.1(B:O) S1.4(A:O) S2.1(B:O) S2.4(A:O)

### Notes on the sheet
- 1 | PRODUCTION | MIKE P.
- Fault LED Indication
- CTRL Switches | Address Select Jumpers
- RUN
- Low
- OFF
- DNI
- Low
- RUN
- OFF
- Low
- Install R21 to allow one switch to control all channels.
  One RUN switch set to 'off' will disable all channels.
- PWRGD Indicator
- Float
- WDI/RESETB Pushbutton
- RESET | Low
- Write-Protect
- High
- Off
- On
- MIKE P.
- NOTES: UNLESS OTHERWISE SPECIFIED:
- MIKE P.
- 1. ALL RESISTORS ARE 1% 0603.
- 24-CHANNEL Digital PSM Board
  that Controls 3 DC1361B Boards
- 2. ALL CAPACITORS ARE 0603.
- LTC2980-24
- DEMO CIRCUIT 3094A | 1

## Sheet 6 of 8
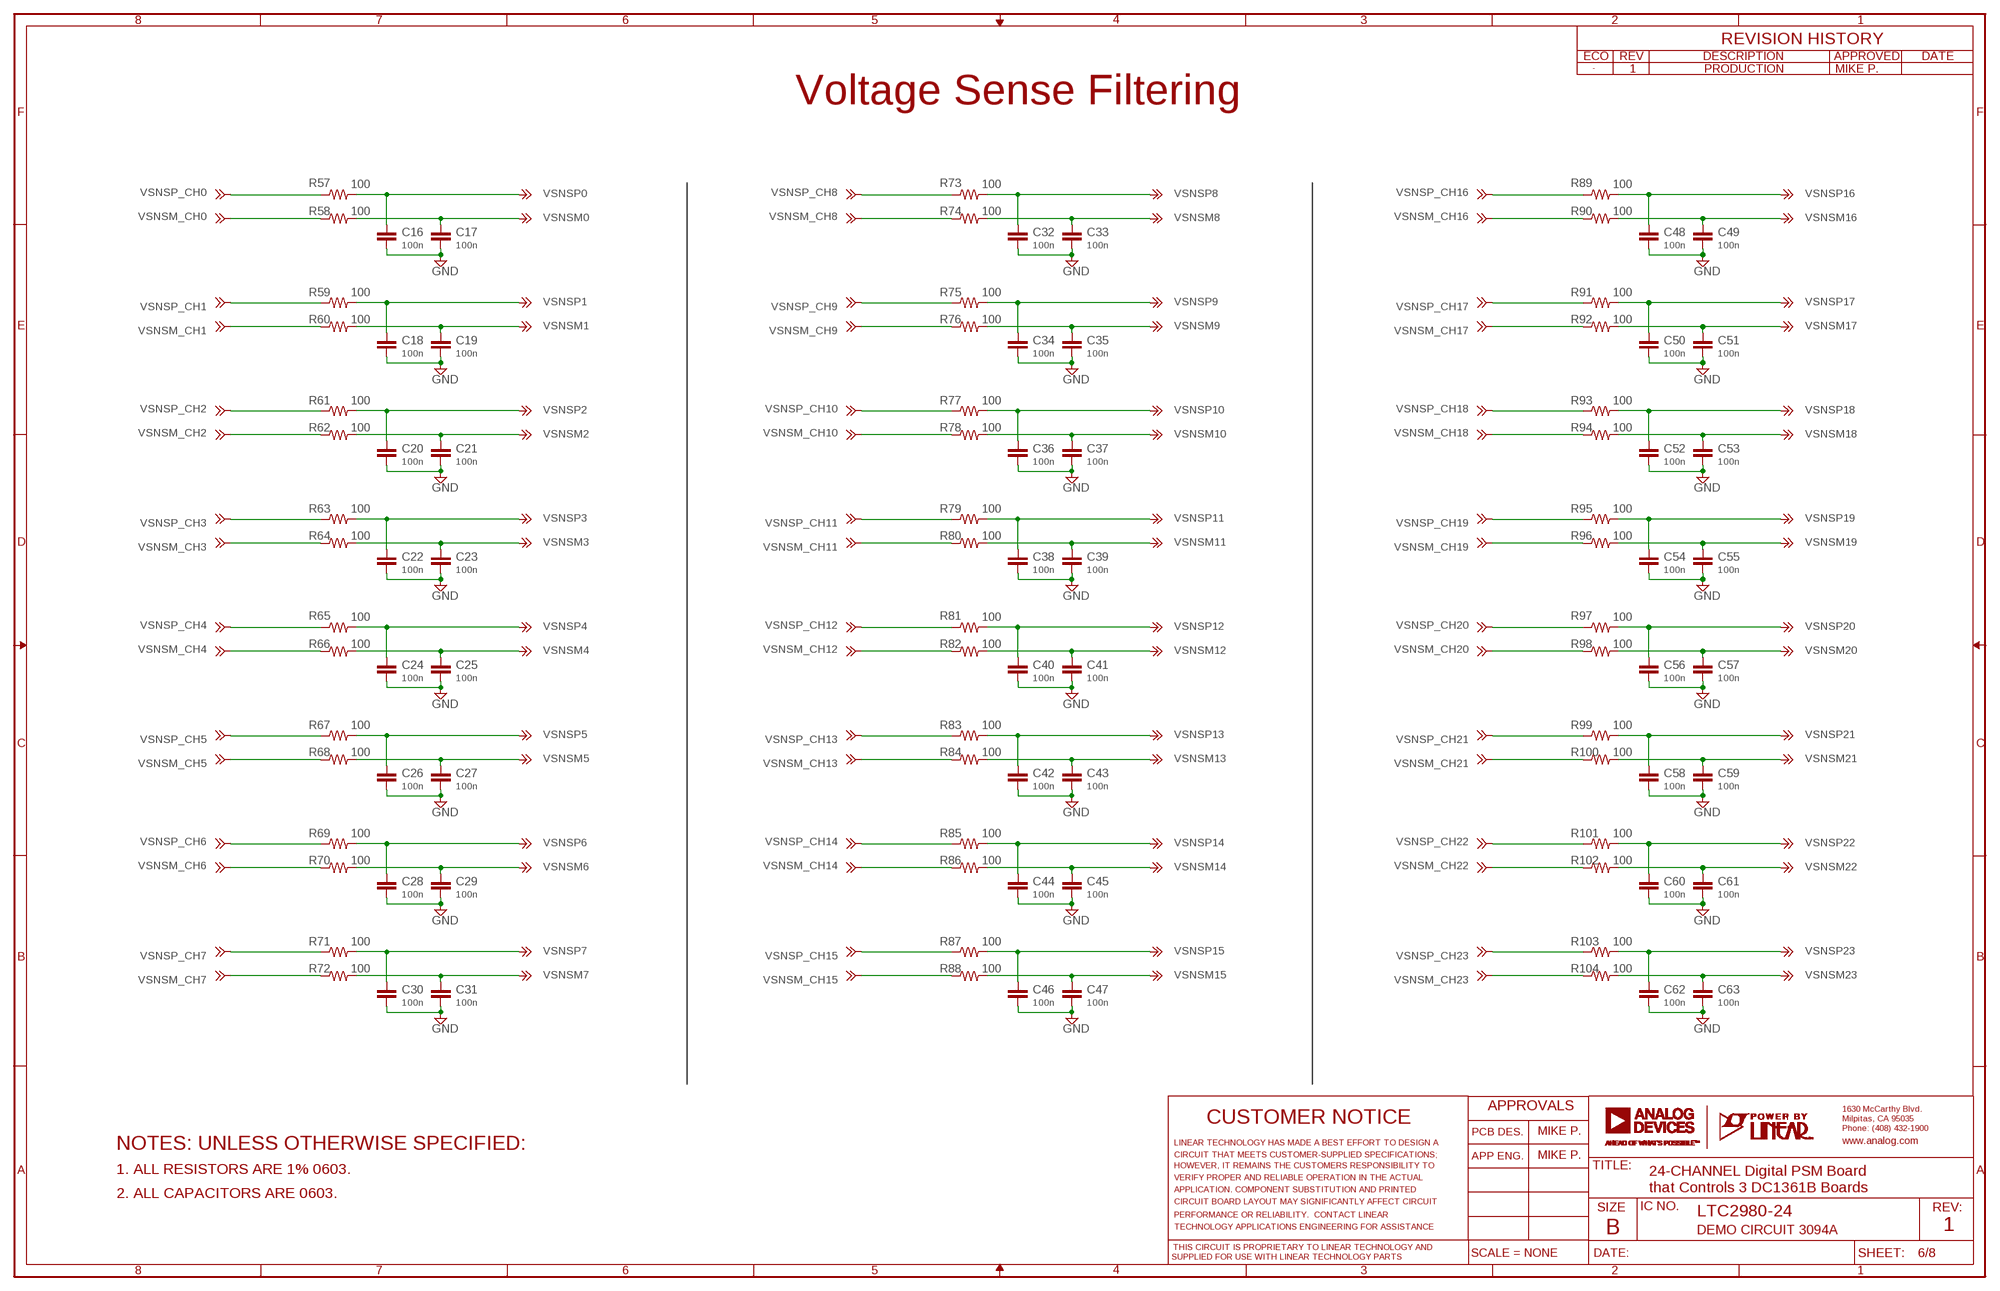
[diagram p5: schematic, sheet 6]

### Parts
C16  100n  CC0603_BOX  [C0603_BOX]
C17  100n  CC0603_BOX  [C0603_BOX]
C18  100n  CC0603_BOX  [C0603_BOX]
C19  100n  CC0603_BOX  [C0603_BOX]
C20  100n  CC0603_BOX  [C0603_BOX]
C21  100n  CC0603_BOX  [C0603_BOX]
C22  100n  CC0603_BOX  [C0603_BOX]
C23  100n  CC0603_BOX  [C0603_BOX]
C24  100n  CC0603_BOX  [C0603_BOX]
C25  100n  CC0603_BOX  [C0603_BOX]
C26  100n  CC0603_BOX  [C0603_BOX]
C27  100n  CC0603_BOX  [C0603_BOX]
C28  100n  CC0603_BOX  [C0603_BOX]
C29  100n  CC0603_BOX  [C0603_BOX]
C30  100n  CC0603_BOX  [C0603_BOX]
C31  100n  CC0603_BOX  [C0603_BOX]
C32  100n  CC0603_BOX  [C0603_BOX]
C33  100n  CC0603_BOX  [C0603_BOX]
C34  100n  CC0603_BOX  [C0603_BOX]
C35  100n  CC0603_BOX  [C0603_BOX]
C36  100n  CC0603_BOX  [C0603_BOX]
C37  100n  CC0603_BOX  [C0603_BOX]
C38  100n  CC0603_BOX  [C0603_BOX]
C39  100n  CC0603_BOX  [C0603_BOX]
C40  100n  CC0603_BOX  [C0603_BOX]
C41  100n  CC0603_BOX  [C0603_BOX]
C42  100n  CC0603_BOX  [C0603_BOX]
C43  100n  CC0603_BOX  [C0603_BOX]
C44  100n  CC0603_BOX  [C0603_BOX]
C45  100n  CC0603_BOX  [C0603_BOX]
C46  100n  CC0603_BOX  [C0603_BOX]
C47  100n  CC0603_BOX  [C0603_BOX]
C48  100n  CC0603_BOX  [C0603_BOX]
C49  100n  CC0603_BOX  [C0603_BOX]
C50  100n  CC0603_BOX  [C0603_BOX]
C51  100n  CC0603_BOX  [C0603_BOX]
C52  100n  CC0603_BOX  [C0603_BOX]
C53  100n  CC0603_BOX  [C0603_BOX]
C54  100n  CC0603_BOX  [C0603_BOX]
C55  100n  CC0603_BOX  [C0603_BOX]
C56  100n  CC0603_BOX  [C0603_BOX]
C57  100n  CC0603_BOX  [C0603_BOX]
C58  100n  CC0603_BOX  [C0603_BOX]
C59  100n  CC0603_BOX  [C0603_BOX]
C60  100n  CC0603_BOX  [C0603_BOX]
C61  100n  CC0603_BOX  [C0603_BOX]
C62  100n  CC0603_BOX  [C0603_BOX]
C63  100n  CC0603_BOX  [C0603_BOX]
R57  100  RR0603_BOX  [R0603_BOX]
R58  100  RR0603_BOX  [R0603_BOX]
R59  100  RR0603_BOX  [R0603_BOX]
R60  100  RR0603_BOX  [R0603_BOX]
R61  100  RR0603_BOX  [R0603_BOX]
R62  100  RR0603_BOX  [R0603_BOX]
R63  100  RR0603_BOX  [R0603_BOX]
R64  100  RR0603_BOX  [R0603_BOX]
R65  100  RR0603_BOX  [R0603_BOX]
R66  100  RR0603_BOX  [R0603_BOX]
R67  100  RR0603_BOX  [R0603_BOX]
R68  100  RR0603_BOX  [R0603_BOX]
R69  100  RR0603_BOX  [R0603_BOX]
R70  100  RR0603_BOX  [R0603_BOX]
R71  100  RR0603_BOX  [R0603_BOX]
R72  100  RR0603_BOX  [R0603_BOX]
R73  100  RR0603_BOX  [R0603_BOX]
R74  100  RR0603_BOX  [R0603_BOX]
R75  100  RR0603_BOX  [R0603_BOX]
R76  100  RR0603_BOX  [R0603_BOX]
R77  100  RR0603_BOX  [R0603_BOX]
R78  100  RR0603_BOX  [R0603_BOX]
R79  100  RR0603_BOX  [R0603_BOX]
R80  100  RR0603_BOX  [R0603_BOX]
R81  100  RR0603_BOX  [R0603_BOX]
R82  100  RR0603_BOX  [R0603_BOX]
R83  100  RR0603_BOX  [R0603_BOX]
R84  100  RR0603_BOX  [R0603_BOX]
R85  100  RR0603_BOX  [R0603_BOX]
R86  100  RR0603_BOX  [R0603_BOX]
R87  100  RR0603_BOX  [R0603_BOX]
R88  100  RR0603_BOX  [R0603_BOX]
R89  100  RR0603_BOX  [R0603_BOX]
R90  100  RR0603_BOX  [R0603_BOX]
R91  100  RR0603_BOX  [R0603_BOX]
R92  100  RR0603_BOX  [R0603_BOX]
R93  100  RR0603_BOX  [R0603_BOX]
R94  100  RR0603_BOX  [R0603_BOX]
R95  100  RR0603_BOX  [R0603_BOX]
R96  100  RR0603_BOX  [R0603_BOX]
R97  100  RR0603_BOX  [R0603_BOX]
R98  100  RR0603_BOX  [R0603_BOX]
R99  100  RR0603_BOX  [R0603_BOX]
R100  100  RR0603_BOX  [R0603_BOX]
R101  100  RR0603_BOX  [R0603_BOX]
R102  100  RR0603_BOX  [R0603_BOX]
R103  100  RR0603_BOX  [R0603_BOX]
R104  100  RR0603_BOX  [R0603_BOX]

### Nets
GND: C16.2 C17.2 C18.2 C19.2 C20.2 C21.2 C22.2 C23.2 C24.2 C25.2 C26.2 C27.2 C28.2 C29.2 C30.2 C31.2 C32.2 C33.2 C34.2 C35.2 C36.2 C37.2 C38.2 C39.2 C40.2 C41.2 C42.2 C43.2 C44.2 C45.2 C46.2 C47.2 C48.2 C49.2 C50.2 C51.2 C52.2 C53.2 C54.2 C55.2 C56.2 C57.2 C58.2 C59.2 C60.2 C61.2 C62.2 C63.2 ; also sheet 2,3,4,5,7,8
VSNSM0: C17.1 R58.2 ; also sheet 2
VSNSM1: C19.1 R60.2 ; also sheet 2
VSNSM2: C21.1 R62.2 ; also sheet 2
VSNSM3: C23.1 R64.2 ; also sheet 2
VSNSM4: C25.1 R66.2 ; also sheet 2
VSNSM5: C27.1 R68.2 ; also sheet 2
VSNSM6: C29.1 R70.2 ; also sheet 2
VSNSM7: C31.1 R72.2 ; also sheet 2
VSNSM8: C33.1 R74.2 ; also sheet 3
VSNSM9: C35.1 R76.2 ; also sheet 3
VSNSM10: C37.1 R78.2 ; also sheet 3
VSNSM11: C39.1 R80.2 ; also sheet 3
VSNSM12: C41.1 R82.2 ; also sheet 3
VSNSM13: C43.1 R84.2 ; also sheet 3
VSNSM14: C45.1 R86.2 ; also sheet 3
VSNSM15: C47.1 R88.2 ; also sheet 3
VSNSM16: C49.1 R90.2 ; also sheet 4
VSNSM17: C51.1 R92.2 ; also sheet 4
VSNSM18: C53.1 R94.2 ; also sheet 4
VSNSM19: C55.1 R96.2 ; also sheet 4
VSNSM20: C57.1 R98.2 ; also sheet 4
VSNSM21: C59.1 R100.2 ; also sheet 4
VSNSM22: C61.1 R102.2 ; also sheet 4
VSNSM23: C63.1 R104.2 ; also sheet 4
VSNSM_CH0: R58.1 ; also sheet 7
VSNSM_CH1: R60.1 ; also sheet 7
VSNSM_CH2: R62.1 ; also sheet 7
VSNSM_CH3: R64.1 ; also sheet 7
VSNSM_CH4: R66.1 ; also sheet 7
VSNSM_CH5: R68.1 ; also sheet 7
VSNSM_CH6: R70.1 ; also sheet 7
VSNSM_CH7: R72.1 ; also sheet 7
VSNSM_CH8: R74.1 ; also sheet 7
VSNSM_CH9: R76.1 ; also sheet 7
VSNSM_CH10: R78.1 ; also sheet 7
VSNSM_CH11: R80.1 ; also sheet 7
VSNSM_CH12: R82.1 ; also sheet 7
VSNSM_CH13: R84.1 ; also sheet 7
VSNSM_CH14: R86.1 ; also sheet 7
VSNSM_CH15: R88.1 ; also sheet 7
VSNSM_CH16: R90.1 ; also sheet 7
VSNSM_CH17: R92.1 ; also sheet 7
VSNSM_CH18: R94.1 ; also sheet 7
VSNSM_CH19: R96.1 ; also sheet 7
VSNSM_CH20: R98.1 ; also sheet 7
VSNSM_CH21: R100.1 ; also sheet 7
VSNSM_CH22: R102.1 ; also sheet 7
VSNSM_CH23: R104.1 ; also sheet 7
VSNSP0: C16.1 R57.2 ; also sheet 2
VSNSP1: C18.1 R59.2 ; also sheet 2
VSNSP2: C20.1 R61.2 ; also sheet 2
VSNSP3: C22.1 R63.2 ; also sheet 2
VSNSP4: C24.1 R65.2 ; also sheet 2
VSNSP5: C26.1 R67.2 ; also sheet 2
VSNSP6: C28.1 R69.2 ; also sheet 2
VSNSP7: C30.1 R71.2 ; also sheet 2
VSNSP8: C32.1 R73.2 ; also sheet 3
VSNSP9: C34.1 R75.2 ; also sheet 3
VSNSP10: C36.1 R77.2 ; also sheet 3
VSNSP11: C38.1 R79.2 ; also sheet 3
VSNSP12: C40.1 R81.2 ; also sheet 3
VSNSP13: C42.1 R83.2 ; also sheet 3
VSNSP14: C44.1 R85.2 ; also sheet 3
VSNSP15: C46.1 R87.2 ; also sheet 3
VSNSP16: C48.1 R89.2 ; also sheet 4
VSNSP17: C50.1 R91.2 ; also sheet 4
VSNSP18: C52.1 R93.2 ; also sheet 4
VSNSP19: C54.1 R95.2 ; also sheet 4
VSNSP20: C56.1 R97.2 ; also sheet 4
VSNSP21: C58.1 R99.2 ; also sheet 4
VSNSP22: C60.1 R101.2 ; also sheet 4
VSNSP23: C62.1 R103.2 ; also sheet 4
VSNSP_CH0: R57.1 ; also sheet 7
VSNSP_CH1: R59.1 ; also sheet 7
VSNSP_CH2: R61.1 ; also sheet 7
VSNSP_CH3: R63.1 ; also sheet 7
VSNSP_CH4: R65.1 ; also sheet 7
VSNSP_CH5: R67.1 ; also sheet 7
VSNSP_CH6: R69.1 ; also sheet 7
VSNSP_CH7: R71.1 ; also sheet 7
VSNSP_CH8: R73.1 ; also sheet 7
VSNSP_CH9: R75.1 ; also sheet 7
VSNSP_CH10: R77.1 ; also sheet 7
VSNSP_CH11: R79.1 ; also sheet 7
VSNSP_CH12: R81.1 ; also sheet 7
VSNSP_CH13: R83.1 ; also sheet 7
VSNSP_CH14: R85.1 ; also sheet 7
VSNSP_CH15: R87.1 ; also sheet 7
VSNSP_CH16: R89.1 ; also sheet 7
VSNSP_CH17: R91.1 ; also sheet 7
VSNSP_CH18: R93.1 ; also sheet 7
VSNSP_CH19: R95.1 ; also sheet 7
VSNSP_CH20: R97.1 ; also sheet 7
VSNSP_CH21: R99.1 ; also sheet 7
VSNSP_CH22: R101.1 ; also sheet 7
VSNSP_CH23: R103.1 ; also sheet 7

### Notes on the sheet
- 1 | PRODUCTION | MIKE P.
- Voltage Sense Filtering
- MIKE P.
- NOTES: UNLESS OTHERWISE SPECIFIED:
- MIKE P.
- 1. ALL RESISTORS ARE 1% 0603.
- 24-CHANNEL Digital PSM Board
  that Controls 3 DC1361B Boards
- 2. ALL CAPACITORS ARE 0603.
- LTC2980-24
- DEMO CIRCUIT 3094A | 1

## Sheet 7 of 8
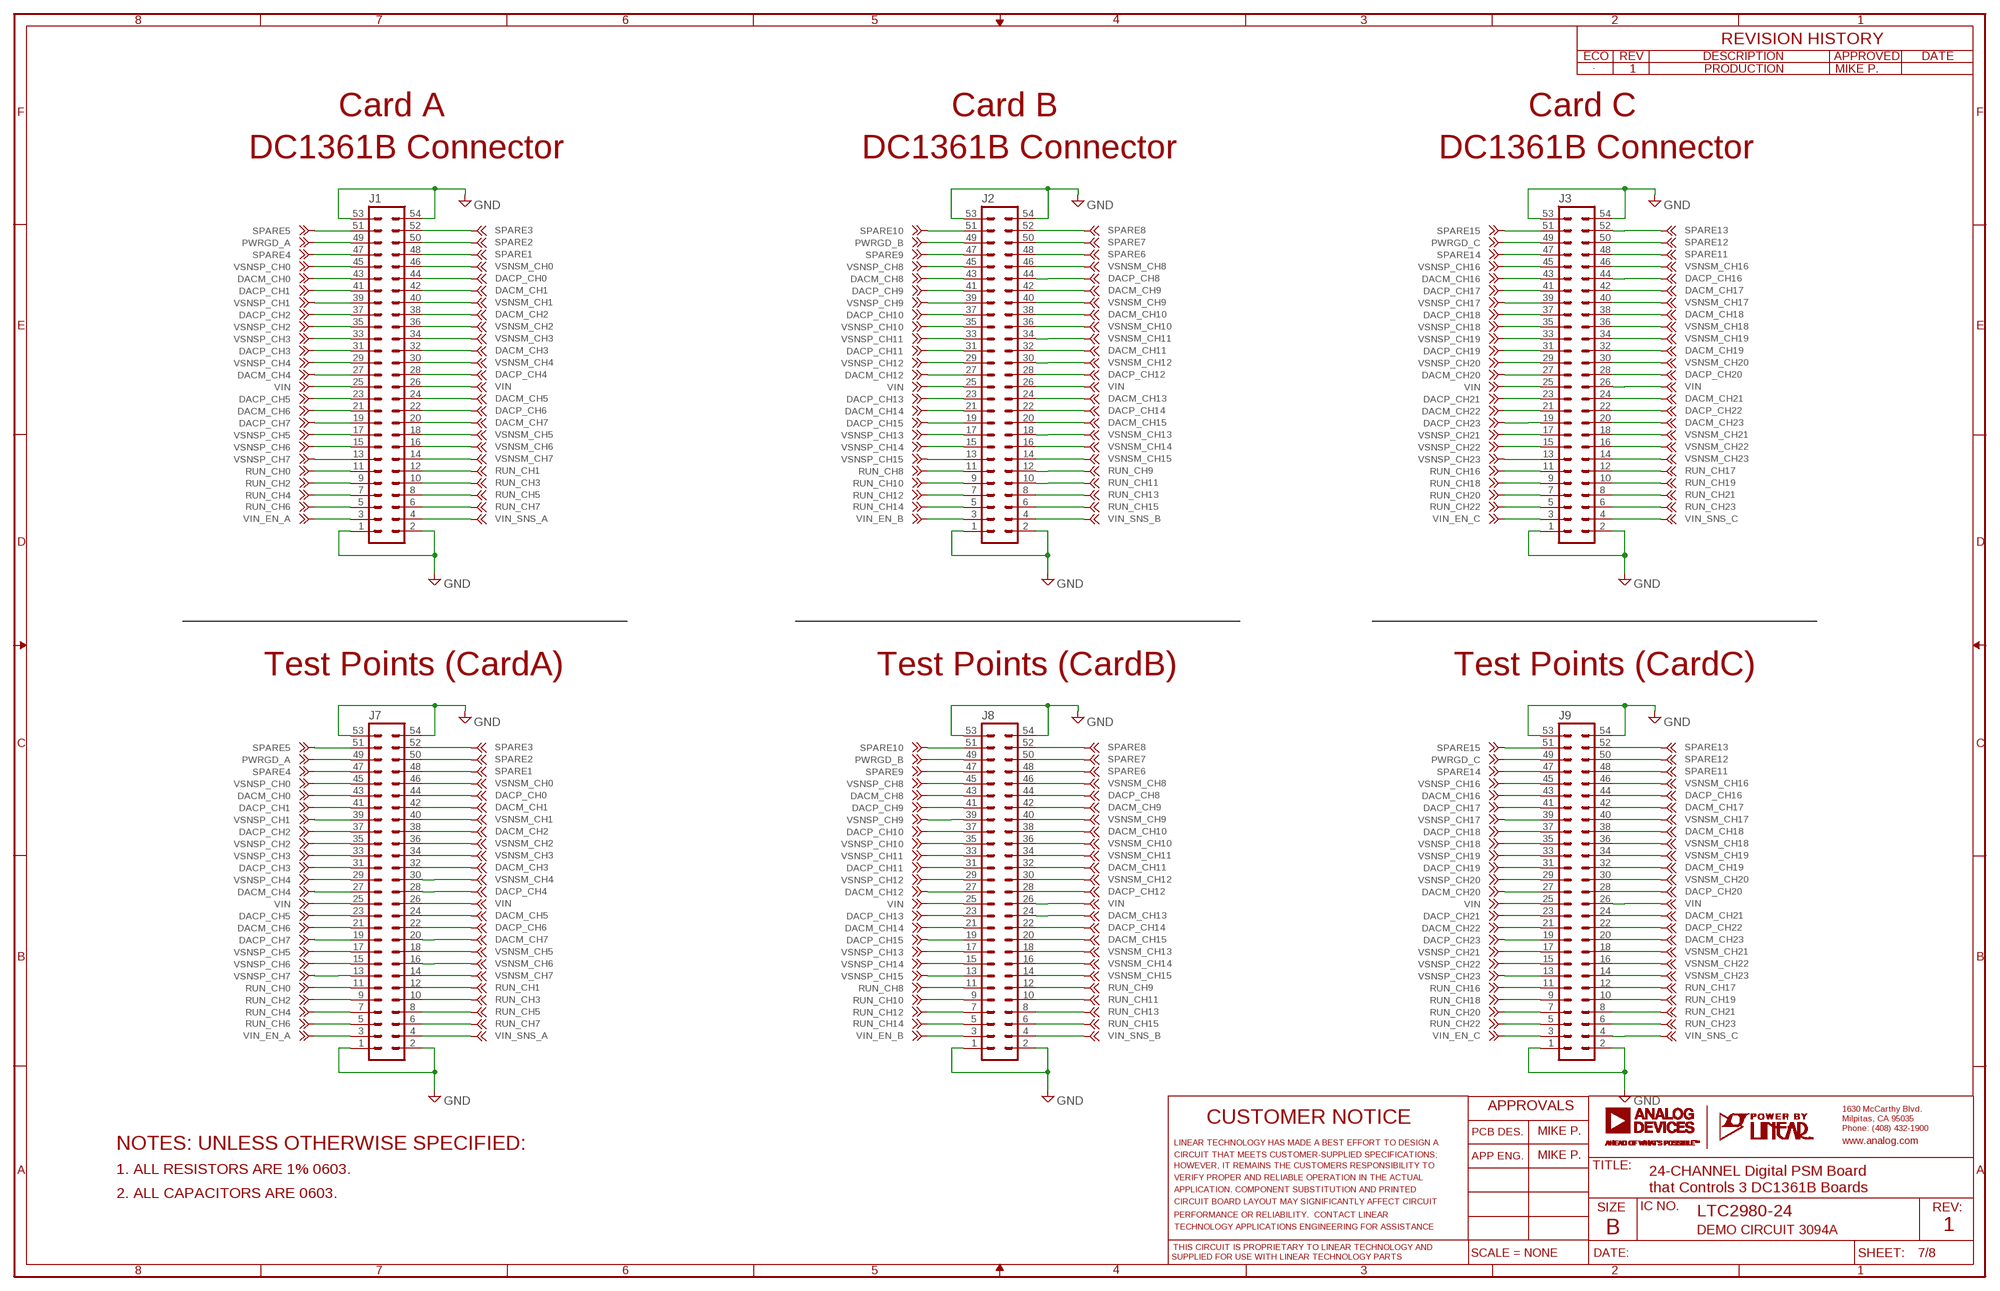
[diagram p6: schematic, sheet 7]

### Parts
J1  CONN_2X27F  [PINHEAD_2X27_RECEPTACLE]
J2  CONN_2X27F  [PINHEAD_2X27_RECEPTACLE]
J3  CONN_2X27F  [PINHEAD_2X27_RECEPTACLE]
J7  CONN_2X27_NO_SILK  [PINHEAD_2X27_RECEPTACLE_NO_SILK]
J8  CONN_2X27_NO_SILK  [PINHEAD_2X27_RECEPTACLE_NO_SILK]
J9  CONN_2X27_NO_SILK  [PINHEAD_2X27_RECEPTACLE_NO_SILK]

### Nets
DACM_CH0: J1.43 J7.43
DACM_CH1: J1.42 J7.42
DACM_CH2: J1.38 J7.38
DACM_CH3: J1.32 J7.32
DACM_CH4: J1.27 J7.27
DACM_CH5: J1.24 J7.24
DACM_CH6: J1.21 J7.21
DACM_CH7: J1.20 J7.20
DACM_CH8: J2.43 J8.43
DACM_CH9: J2.42 J8.42
DACM_CH10: J2.38 J8.38
DACM_CH11: J2.32 J8.32
DACM_CH12: J2.27 J8.27
DACM_CH13: J2.24 J8.24
DACM_CH14: J2.21 J8.21
DACM_CH15: J2.20 J8.20
DACM_CH16: J3.43 J9.43
DACM_CH17: J3.42 J9.42
DACM_CH18: J3.38 J9.38
DACM_CH19: J3.32 J9.32
DACM_CH20: J3.27 J9.27
DACM_CH21: J3.24 J9.24
DACM_CH22: J3.21 J9.21
DACM_CH23: J3.20 J9.20
DACP_CH0: J1.44 J7.44 ; also sheet 2
DACP_CH1: J1.41 J7.41 ; also sheet 2
DACP_CH2: J1.37 J7.37 ; also sheet 2
DACP_CH3: J1.31 J7.31 ; also sheet 2
DACP_CH4: J1.28 J7.28 ; also sheet 2
DACP_CH5: J1.23 J7.23 ; also sheet 2
DACP_CH6: J1.22 J7.22 ; also sheet 2
DACP_CH7: J1.19 J7.19 ; also sheet 2
DACP_CH8: J2.44 J8.44 ; also sheet 3
DACP_CH9: J2.41 J8.41 ; also sheet 3
DACP_CH10: J2.37 J8.37 ; also sheet 3
DACP_CH11: J2.31 J8.31 ; also sheet 3
DACP_CH12: J2.28 J8.28 ; also sheet 3
DACP_CH13: J2.23 J8.23 ; also sheet 3
DACP_CH14: J2.22 J8.22 ; also sheet 3
DACP_CH15: J2.19 J8.19 ; also sheet 3
DACP_CH16: J3.44 J9.44 ; also sheet 4
DACP_CH17: J3.41 J9.41 ; also sheet 4
DACP_CH18: J3.37 J9.37 ; also sheet 4
DACP_CH19: J3.31 J9.31 ; also sheet 4
DACP_CH20: J3.28 J9.28 ; also sheet 4
DACP_CH21: J3.23 J9.23 ; also sheet 4
DACP_CH22: J3.22 J9.22 ; also sheet 4
DACP_CH23: J3.19 J9.19 ; also sheet 4
GND: J1.1 J1.2 J1.53 J1.54 J2.1 J2.2 J2.53 J2.54 J3.1 J3.2 J3.53 J3.54 J7.1 J7.2 J7.53 J7.54 J8.1 J8.2 J8.53 J8.54 J9.1 J9.2 J9.53 J9.54 ; also sheet 2,3,4,5,6,8
PWRGD_A: J1.49 J7.49
PWRGD_B: J2.49 J8.49
PWRGD_C: J3.49 J9.49
RUN_CH0: J1.11 J7.11 ; also sheet 2
RUN_CH1: J1.12 J7.12 ; also sheet 2
RUN_CH2: J1.9 J7.9 ; also sheet 2
RUN_CH3: J1.10 J7.10 ; also sheet 2
RUN_CH4: J1.7 J7.7 ; also sheet 2
RUN_CH5: J1.8 J7.8 ; also sheet 2
RUN_CH6: J1.5 J7.5 ; also sheet 2
RUN_CH7: J1.6 J7.6 ; also sheet 2
RUN_CH8: J2.11 J8.11 ; also sheet 3
RUN_CH9: J2.12 J8.12 ; also sheet 3
RUN_CH10: J2.9 J8.9 ; also sheet 3
RUN_CH11: J2.10 J8.10 ; also sheet 3
RUN_CH12: J2.7 J8.7 ; also sheet 3
RUN_CH13: J2.8 J8.8 ; also sheet 3
RUN_CH14: J2.5 J8.5 ; also sheet 3
RUN_CH15: J2.6 J8.6 ; also sheet 3
RUN_CH16: J3.11 J9.11 ; also sheet 4
RUN_CH17: J3.12 J9.12 ; also sheet 4
RUN_CH18: J3.9 J9.9 ; also sheet 4
RUN_CH19: J3.10 J9.10 ; also sheet 4
RUN_CH20: J3.7 J9.7 ; also sheet 4
RUN_CH21: J3.8 J9.8 ; also sheet 4
RUN_CH22: J3.5 J9.5 ; also sheet 4
RUN_CH23: J3.6 J9.6 ; also sheet 4
SPARE1: J1.48 J7.48
SPARE2: J1.50 J7.50
SPARE3: J1.52 J7.52
SPARE4: J1.47 J7.47 ; also sheet 8
SPARE5: J1.51 J7.51
SPARE6: J2.48 J8.48
SPARE7: J2.50 J8.50
SPARE8: J2.52 J8.52
SPARE9: J2.47 J8.47
SPARE10: J2.51 J8.51
SPARE11: J3.48 J9.48
SPARE12: J3.50 J9.50
SPARE13: J3.52 J9.52
SPARE14: J3.47 J9.47
SPARE15: J3.51 J9.51
VIN: J1.25 J1.26 J2.25 J2.26 J3.25 J3.26 J7.25 J7.26 J8.25 J8.26 J9.25 J9.26 ; also sheet 2,3,4
VIN_EN_A: J1.3 J7.3 ; also sheet 2,8
VIN_EN_B: J2.3 J8.3 ; also sheet 3,8
VIN_EN_C: J3.3 J9.3 ; also sheet 4,8
VIN_SNS_A: J1.4 J7.4 ; also sheet 2,8
VIN_SNS_B: J2.4 J8.4 ; also sheet 3,8
VIN_SNS_C: J3.4 J9.4 ; also sheet 4,8
VSNSM_CH0: J1.46 J7.46 ; also sheet 6
VSNSM_CH1: J1.40 J7.40 ; also sheet 6
VSNSM_CH2: J1.36 J7.36 ; also sheet 6
VSNSM_CH3: J1.34 J7.34 ; also sheet 6
VSNSM_CH4: J1.30 J7.30 ; also sheet 6
VSNSM_CH5: J1.18 J7.18 ; also sheet 6
VSNSM_CH6: J1.16 J7.16 ; also sheet 6
VSNSM_CH7: J1.14 J7.14 ; also sheet 6
VSNSM_CH8: J2.46 J8.46 ; also sheet 6
VSNSM_CH9: J2.40 J8.40 ; also sheet 6
VSNSM_CH10: J2.36 J8.36 ; also sheet 6
VSNSM_CH11: J2.34 J8.34 ; also sheet 6
VSNSM_CH12: J2.30 J8.30 ; also sheet 6
VSNSM_CH13: J2.18 J8.18 ; also sheet 6
VSNSM_CH14: J2.16 J8.16 ; also sheet 6
VSNSM_CH15: J2.14 J8.14 ; also sheet 6
VSNSM_CH16: J3.46 J9.46 ; also sheet 6
VSNSM_CH17: J3.40 J9.40 ; also sheet 6
VSNSM_CH18: J3.36 J9.36 ; also sheet 6
VSNSM_CH19: J3.34 J9.34 ; also sheet 6
VSNSM_CH20: J3.30 J9.30 ; also sheet 6
VSNSM_CH21: J3.18 J9.18 ; also sheet 6
VSNSM_CH22: J3.16 J9.16 ; also sheet 6
VSNSM_CH23: J3.14 J9.14 ; also sheet 6
VSNSP_CH0: J1.45 J7.45 ; also sheet 6
VSNSP_CH1: J1.39 J7.39 ; also sheet 6
VSNSP_CH2: J1.35 J7.35 ; also sheet 6
VSNSP_CH3: J1.33 J7.33 ; also sheet 6
VSNSP_CH4: J1.29 J7.29 ; also sheet 6
VSNSP_CH5: J1.17 J7.17 ; also sheet 6
VSNSP_CH6: J1.15 J7.15 ; also sheet 6
VSNSP_CH7: J1.13 J7.13 ; also sheet 6
VSNSP_CH8: J2.45 J8.45 ; also sheet 6
VSNSP_CH9: J2.39 J8.39 ; also sheet 6
VSNSP_CH10: J2.35 J8.35 ; also sheet 6
VSNSP_CH11: J2.33 J8.33 ; also sheet 6
VSNSP_CH12: J2.29 J8.29 ; also sheet 6
VSNSP_CH13: J2.17 J8.17 ; also sheet 6
VSNSP_CH14: J2.15 J8.15 ; also sheet 6
VSNSP_CH15: J2.13 J8.13 ; also sheet 6
VSNSP_CH16: J3.45 J9.45 ; also sheet 6
VSNSP_CH17: J3.39 J9.39 ; also sheet 6
VSNSP_CH18: J3.35 J9.35 ; also sheet 6
VSNSP_CH19: J3.33 J9.33 ; also sheet 6
VSNSP_CH20: J3.29 J9.29 ; also sheet 6
VSNSP_CH21: J3.17 J9.17 ; also sheet 6
VSNSP_CH22: J3.15 J9.15 ; also sheet 6
VSNSP_CH23: J3.13 J9.13 ; also sheet 6

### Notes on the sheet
- 1 | PRODUCTION | MIKE P.
- Card A | Card B | Card C
- DC1361B Connector | DC1361B Connector | DC1361B Connector
- Test Points (CardA) | Test Points (CardB) | Test Points (CardC)
- MIKE P.
- NOTES: UNLESS OTHERWISE SPECIFIED:
- MIKE P.
- 1. ALL RESISTORS ARE 1% 0603.
- 24-CHANNEL Digital PSM Board
  that Controls 3 DC1361B Boards
- 2. ALL CAPACITORS ARE 0603.
- LTC2980-24
- DEMO CIRCUIT 3094A | 1

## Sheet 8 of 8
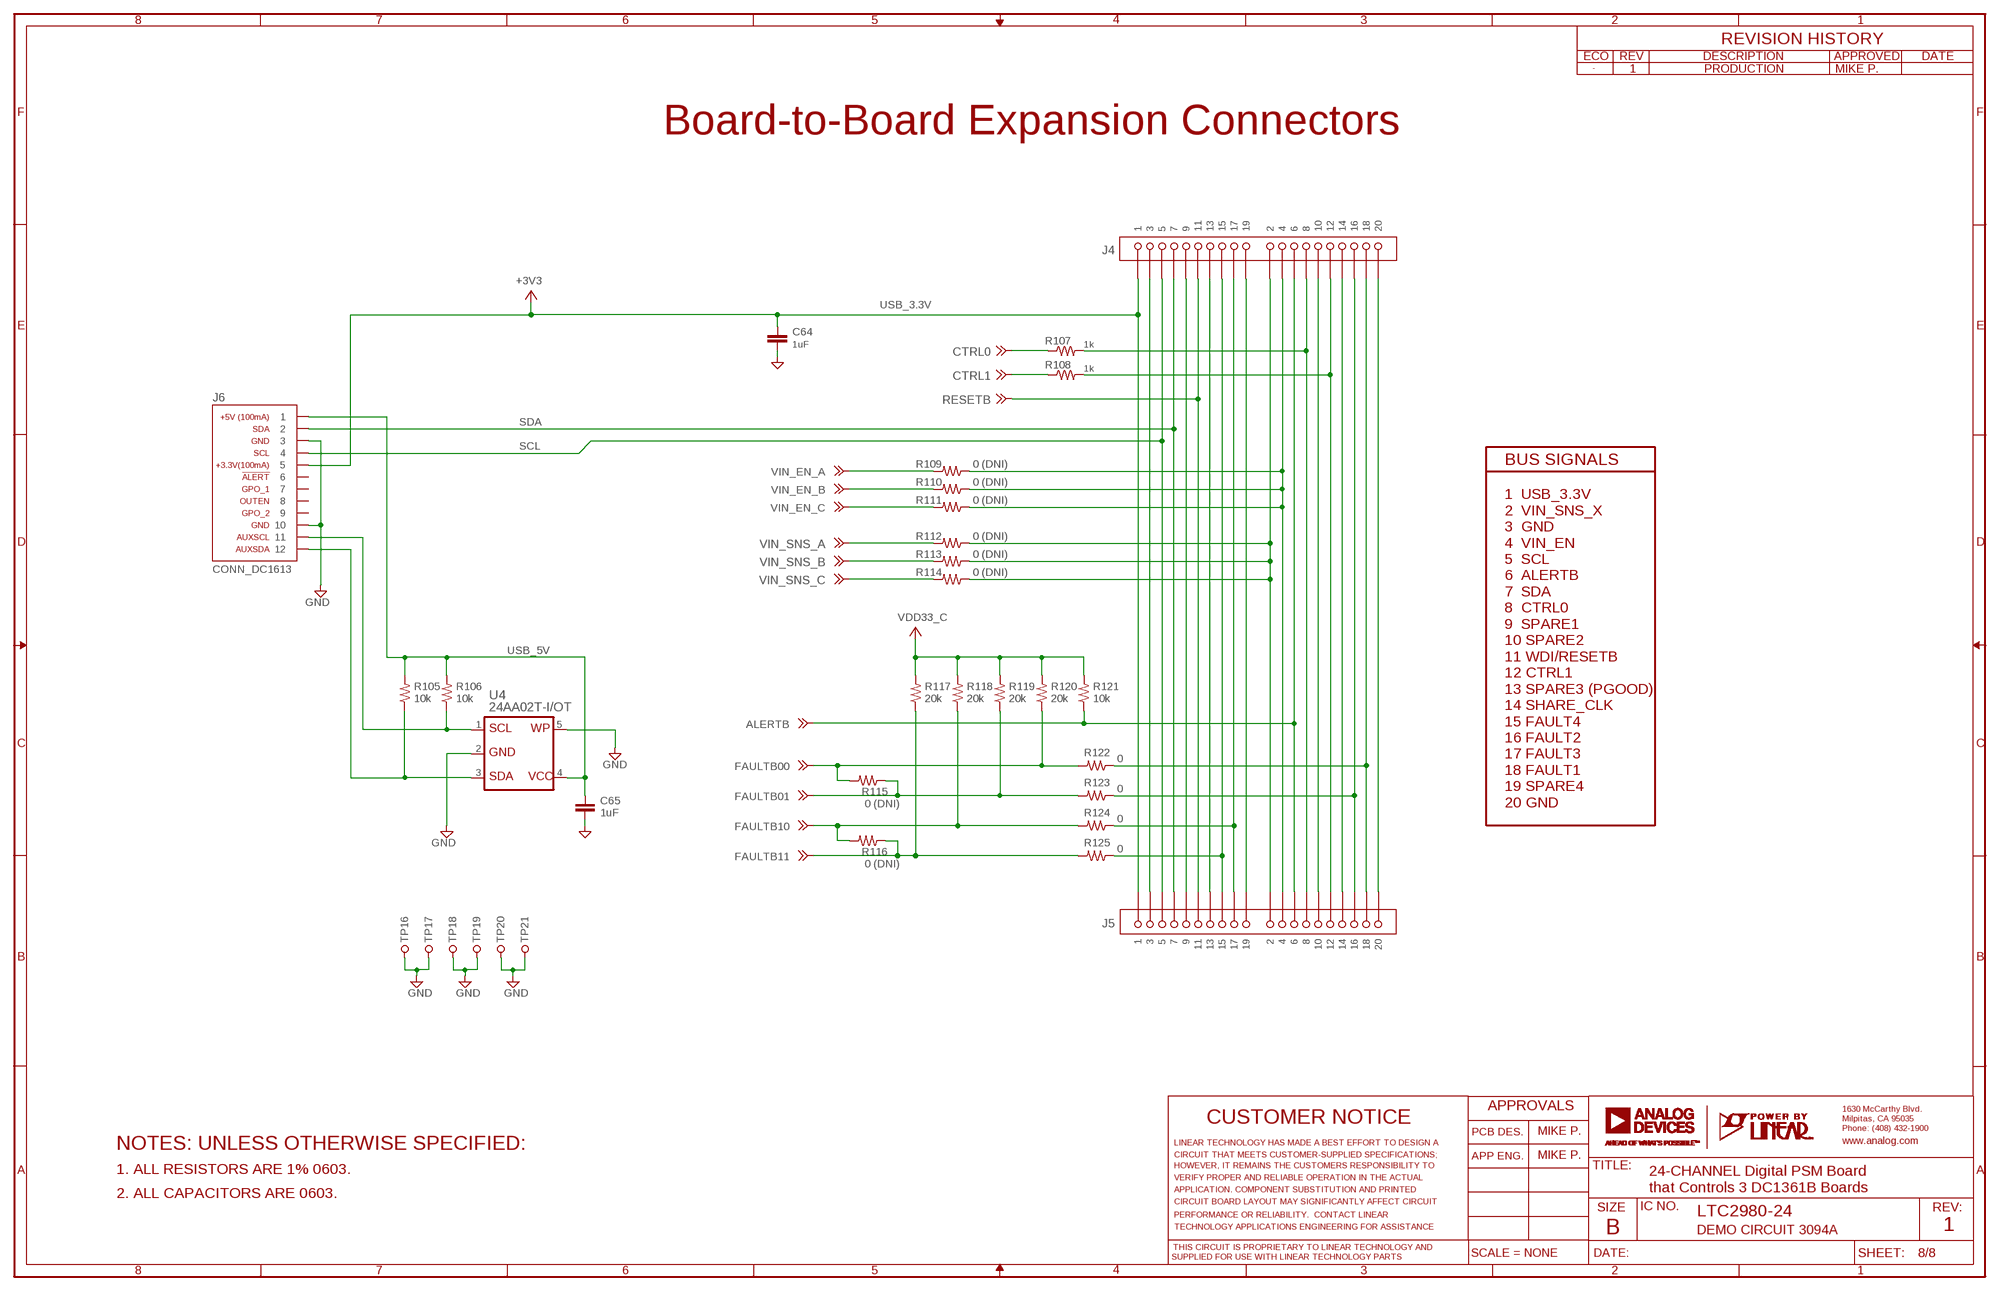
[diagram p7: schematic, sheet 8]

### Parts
C64  1uF  CC0603_BOX  [C0603_BOX]
C65  1uF  CC0603_BOX  [C0603_BOX]
J4  RECEPT_CONN_2X10_0.1INCH  [RECEPT_2X10_0.1INCH]
J5  HEADER_CONN_2X10_0.1INCH  [HEADER_2X10_0.1INCH]
J6  CONN_DC1613  [CONN_DC1613]
R105  10k  RR0603_BOX  [R0603_BOX]
R106  10k  RR0603_BOX  [R0603_BOX]
R107  1k  RR0603_BOX  [R0603_BOX]
R108  1k  RR0603_BOX  [R0603_BOX]
R109  0 (DNI)  RR0603_BOX  [R0603_BOX]
R110  0 (DNI)  RR0603_BOX  [R0603_BOX]
R111  0 (DNI)  RR0603_BOX  [R0603_BOX]
R112  0 (DNI)  RR0603_BOX  [R0603_BOX]
R113  0 (DNI)  RR0603_BOX  [R0603_BOX]
R114  0 (DNI)  RR0603_BOX  [R0603_BOX]
R115  0 (DNI)  RR0603_BOX  [R0603_BOX]
R116  0 (DNI)  RR0603_BOX  [R0603_BOX]
R117  20k  RR0603_BOX  [R0603_BOX]
R118  20k  RR0603_BOX  [R0603_BOX]
R119  20k  RR0603_BOX  [R0603_BOX]
R120  20k  RR0603_BOX  [R0603_BOX]
R121  10k  RR0603_BOX  [R0603_BOX]
R122  0  RR0603_BOX  [R0603_BOX]
R123  0  RR0603_BOX  [R0603_BOX]
R124  0  RR0603_BOX  [R0603_BOX]
R125  0  RR0603_BOX  [R0603_BOX]
TP16  TURRET_LARGE_2501  [TURRET_LARGE_2501]
TP17  TURRET_LARGE_2501  [TURRET_LARGE_2501]
TP18  TURRET_LARGE_2501  [TURRET_LARGE_2501]
TP19  TURRET_LARGE_2501  [TURRET_LARGE_2501]
TP20  TURRET_LARGE_2501  [TURRET_LARGE_2501]
TP21  TURRET_LARGE_2501  [TURRET_LARGE_2501]
U4  24AA02T-I/OT  24AA64  [SOT-23-5]

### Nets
ALERTB: J4.P$6 J5.P$6 R121.1 ; also sheet 2,3,4,5
AUX_SCL: J6.11 R106.1 U4.1
AUX_SDA: J6.12 R105.1 U4.3
AUXFAULTB_3V3: J4.P$4 J5.P$4 R109.1 R110.1 R111.1
CTRL0: R107.1 ; also sheet 2,3,4,5
CTRL0_X: J4.P$8 J5.P$8 R107.2
CTRL1: R108.1 ; also sheet 2,3,4,5
CTRL1_X: J4.P$12 J5.P$12 R108.2
CTRL2: J4.P$9 J5.P$9
CTRL3: J4.P$10 J5.P$10
FAULT1: J4.P$18 J5.P$18 R122.1
FAULT2: J4.P$16 J5.P$16 R123.1
FAULT3: J4.P$17 J5.P$17 R124.1
FAULT4: J4.P$15 J5.P$15 R125.1
FAULTB00: R115.2 R120.1 R122.2 ; also sheet 2,3,4,5
FAULTB01: R115.1 R119.1 R123.2 ; also sheet 2,3,4,5
FAULTB10: R116.2 R118.1 R124.2 ; also sheet 2,3,4,5
FAULTB11: R116.1 R117.1 R125.2 ; also sheet 2,3,4,5
GND: C64.2 C65.2 J4.P$3 J4.P$20 J5.P$3 J5.P$20 J6.3 J6.10 TP16.TP TP17.TP TP18.TP TP19.TP TP20.TP TP21.TP U4.2 U4.5 ; also sheet 2,3,4,5,6,7
N$16: J4.P$13
PGOOD3: J5.P$13
RESETB: J4.P$11 J5.P$11 ; also sheet 2,3,4,5
SCL: J4.P$5 J5.P$5 J6.4 ; also sheet 2,3,4
SDA: J4.P$7 J5.P$7 J6.2 ; also sheet 2,3,4
SHARE_CLK: J4.P$14 J5.P$14 ; also sheet 2,3,4
SPARE4: J4.P$19 J5.P$19 ; also sheet 7
USB_3.3V: C64.1 J4.P$1 J5.P$1 J6.5 ; supply symbol labelled +3V3 ; also sheet 2,3,4
USB_5V: C65.1 J6.1 R105.2 R106.2 U4.4
VDD33_C: R117.2 R118.2 R119.2 R120.2 R121.2 ; supply symbol labelled +3V3 ; also sheet 4,5
VIN_EN_A: R109.2 ; also sheet 2,7
VIN_EN_B: R110.2 ; also sheet 3,7
VIN_EN_C: R111.2 ; also sheet 4,7
VIN_SNS_A: R112.2 ; also sheet 2,7
VIN_SNS_B: R113.2 ; also sheet 3,7
VIN_SNS_C: R114.2 ; also sheet 4,7
VIN_SNS_X: J4.P$2 J5.P$2 R112.1 R113.1 R114.1
Unconnected: J6.6 J6.7 J6.8 J6.9

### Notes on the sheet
- 1 | PRODUCTION | MIKE P.
- Board-to-Board Expansion Connectors
- BUS SIGNALS
- 1  USB_3.3V
  2  VIN_SNS_X
  3  GND
  4  VIN_EN
  5  SCL
  6  ALERTB
  7  SDA
  8  CTRL0
  9  SPARE1
  10 SPARE2
  11 WDI/RESETB
  12 CTRL1
  13 SPARE3 (PGOOD)
  14 SHARE_CLK
  15 FAULT4
  16 FAULT2
  17 FAULT3
  18 FAULT1
  19 SPARE4
  20 GND
- MIKE P.
- NOTES: UNLESS OTHERWISE SPECIFIED:
- MIKE P.
- 1. ALL RESISTORS ARE 1% 0603.
- 24-CHANNEL Digital PSM Board
  that Controls 3 DC1361B Boards
- 2. ALL CAPACITORS ARE 0603.
- LTC2980-24
- DEMO CIRCUIT 3094A | 1

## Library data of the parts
C1-C66 = rcl:C: CAPACITOR, European symbol
J1-J3 = pinhead:CONN_2X27
J4 = con-millmax:RECEPT_CONN_2X10_0.1INCH
J5 = con-millmax:HEADER_CONN_2X10_0.1INCH
J6 = con-fci:CONN_DC1613: Connector for LT DC1613 USB Dongle
J7-J9 = pinhead:CONN_2X27_NO_SILK
JP1-JP6 = pinhead:PINHD-1X4-2MM: PIN HEADER
JP7 = pinhead:PINHD-1X3-2MM: PIN HEADER
LED1-LED5 = led:LED-0603: SMD LED in R0603
M1-M3 = transistor-fet:PCH_
M4 = transistor-fet:NCH
R1-R125 = resistor:R: RESISTOR, American symbol
S1 S2 = kalin:JS202011CQN: SLIDING SWITCH Siemens, distributor Buerklin, 11G766
SW1 = kalin:SWITCH_PTS635: PTS635SL25 Surface Mount Tactile Switch
TP1-TP9 TP14-TP21 = testpad:TURRET_LARGE_2501: Large Test Turret Mill Max 2501
TP10-TP13 = testpad:TESTPOINT: Test Point
U1 = linear-technology:LTC2980-24X
U2 U3 = 74xx-little-us:74*1G09: Single AND Gate with Open-Drain Output
U4 = kalin:24AA64: 64Kbit I2C Serial EEPROM in SOT-23-5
